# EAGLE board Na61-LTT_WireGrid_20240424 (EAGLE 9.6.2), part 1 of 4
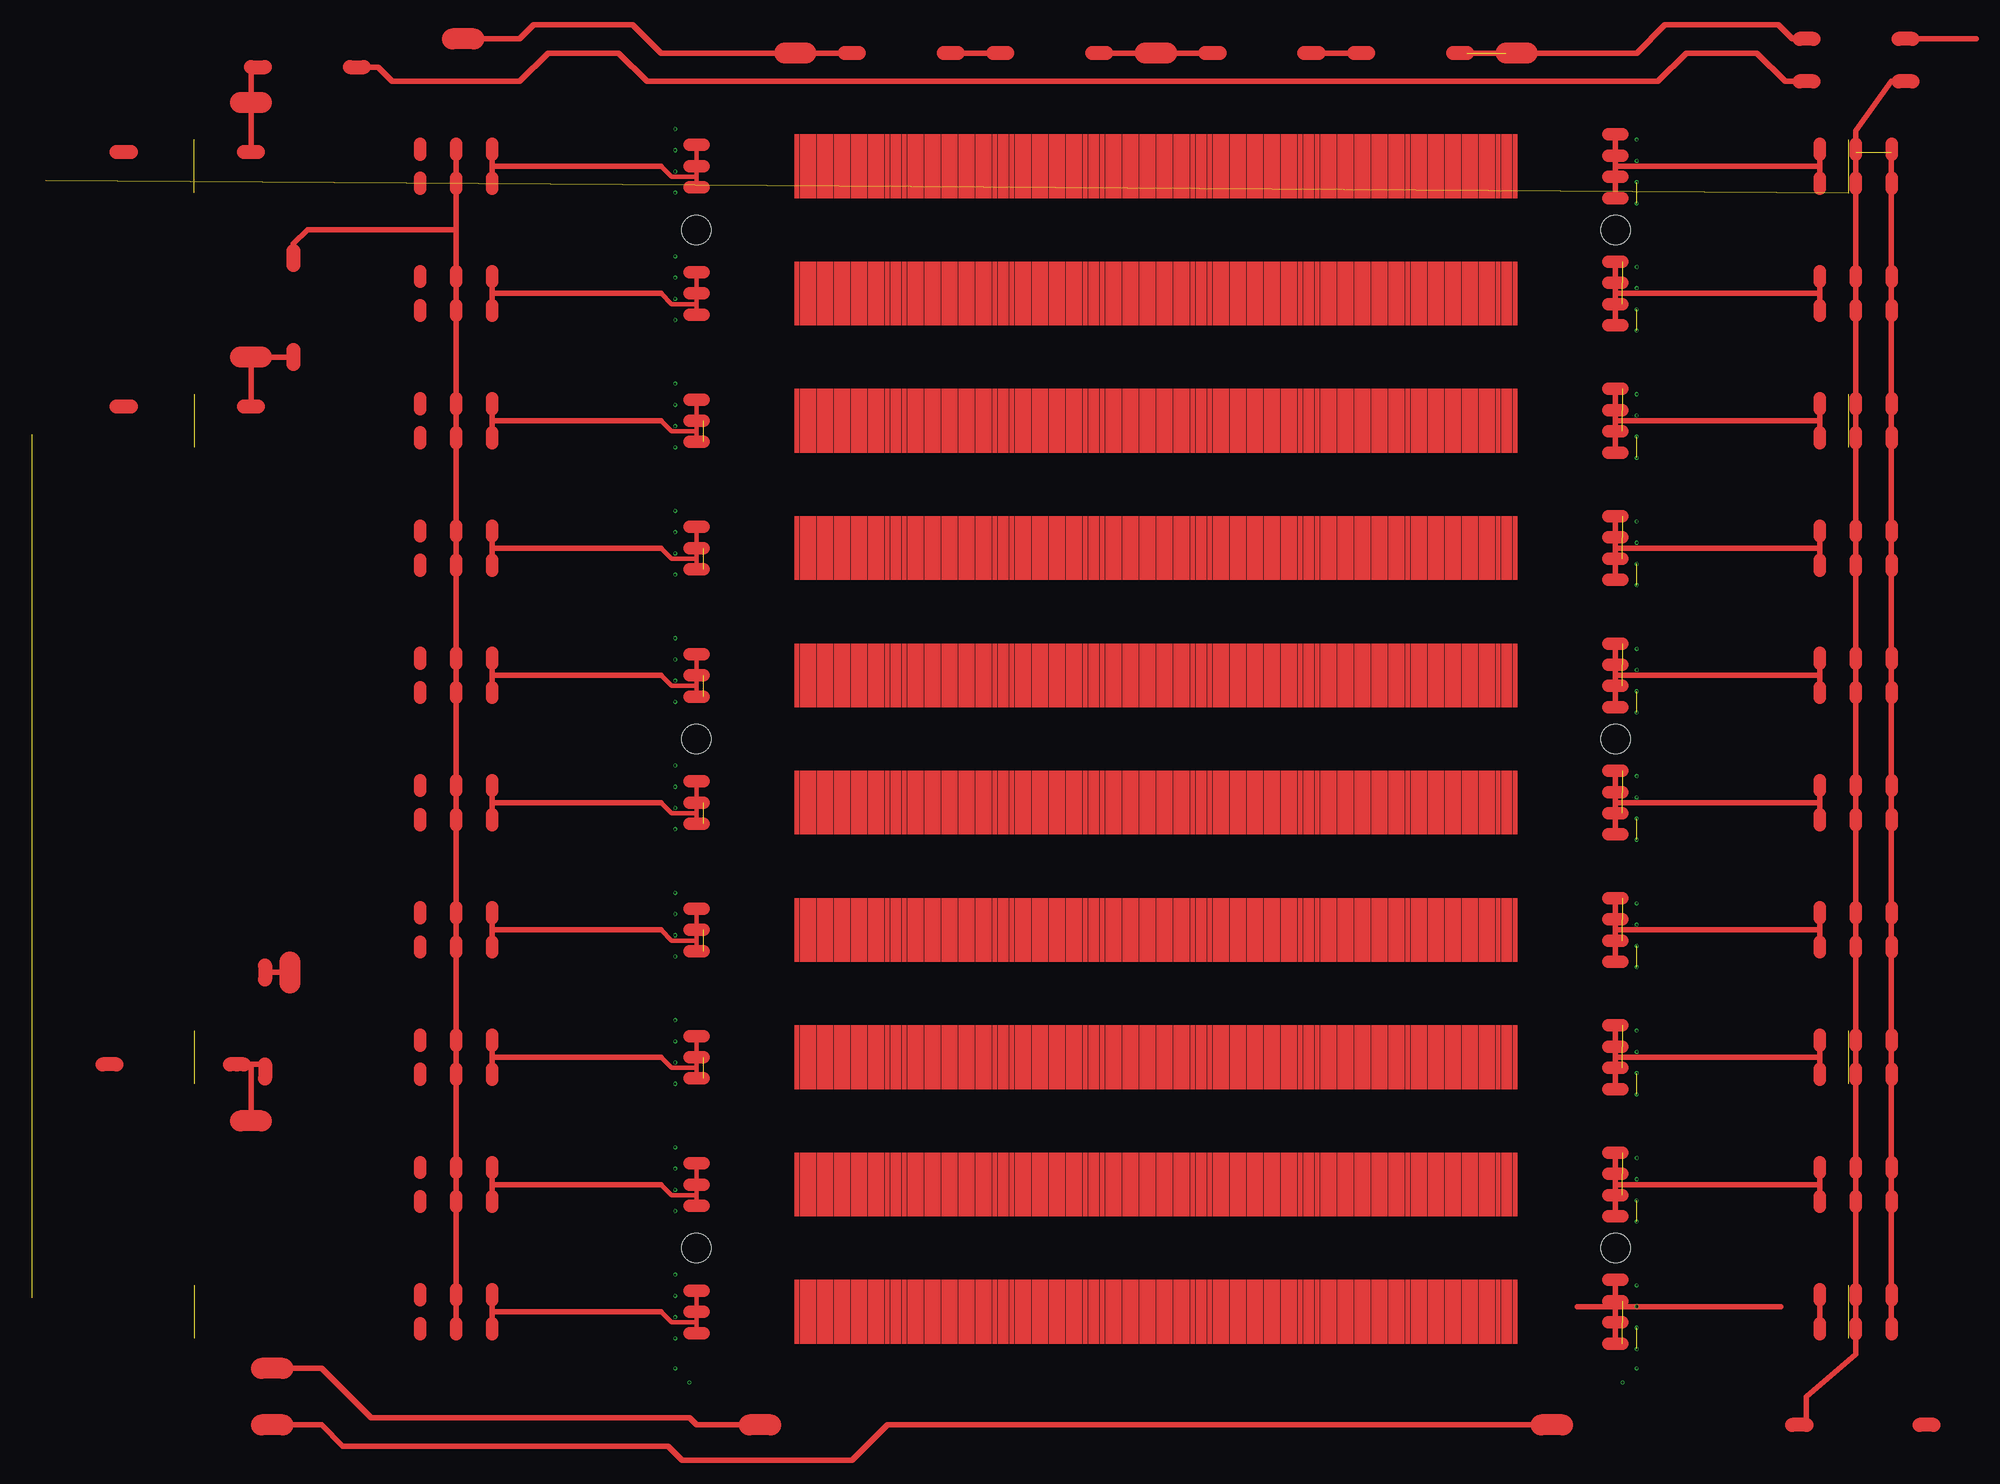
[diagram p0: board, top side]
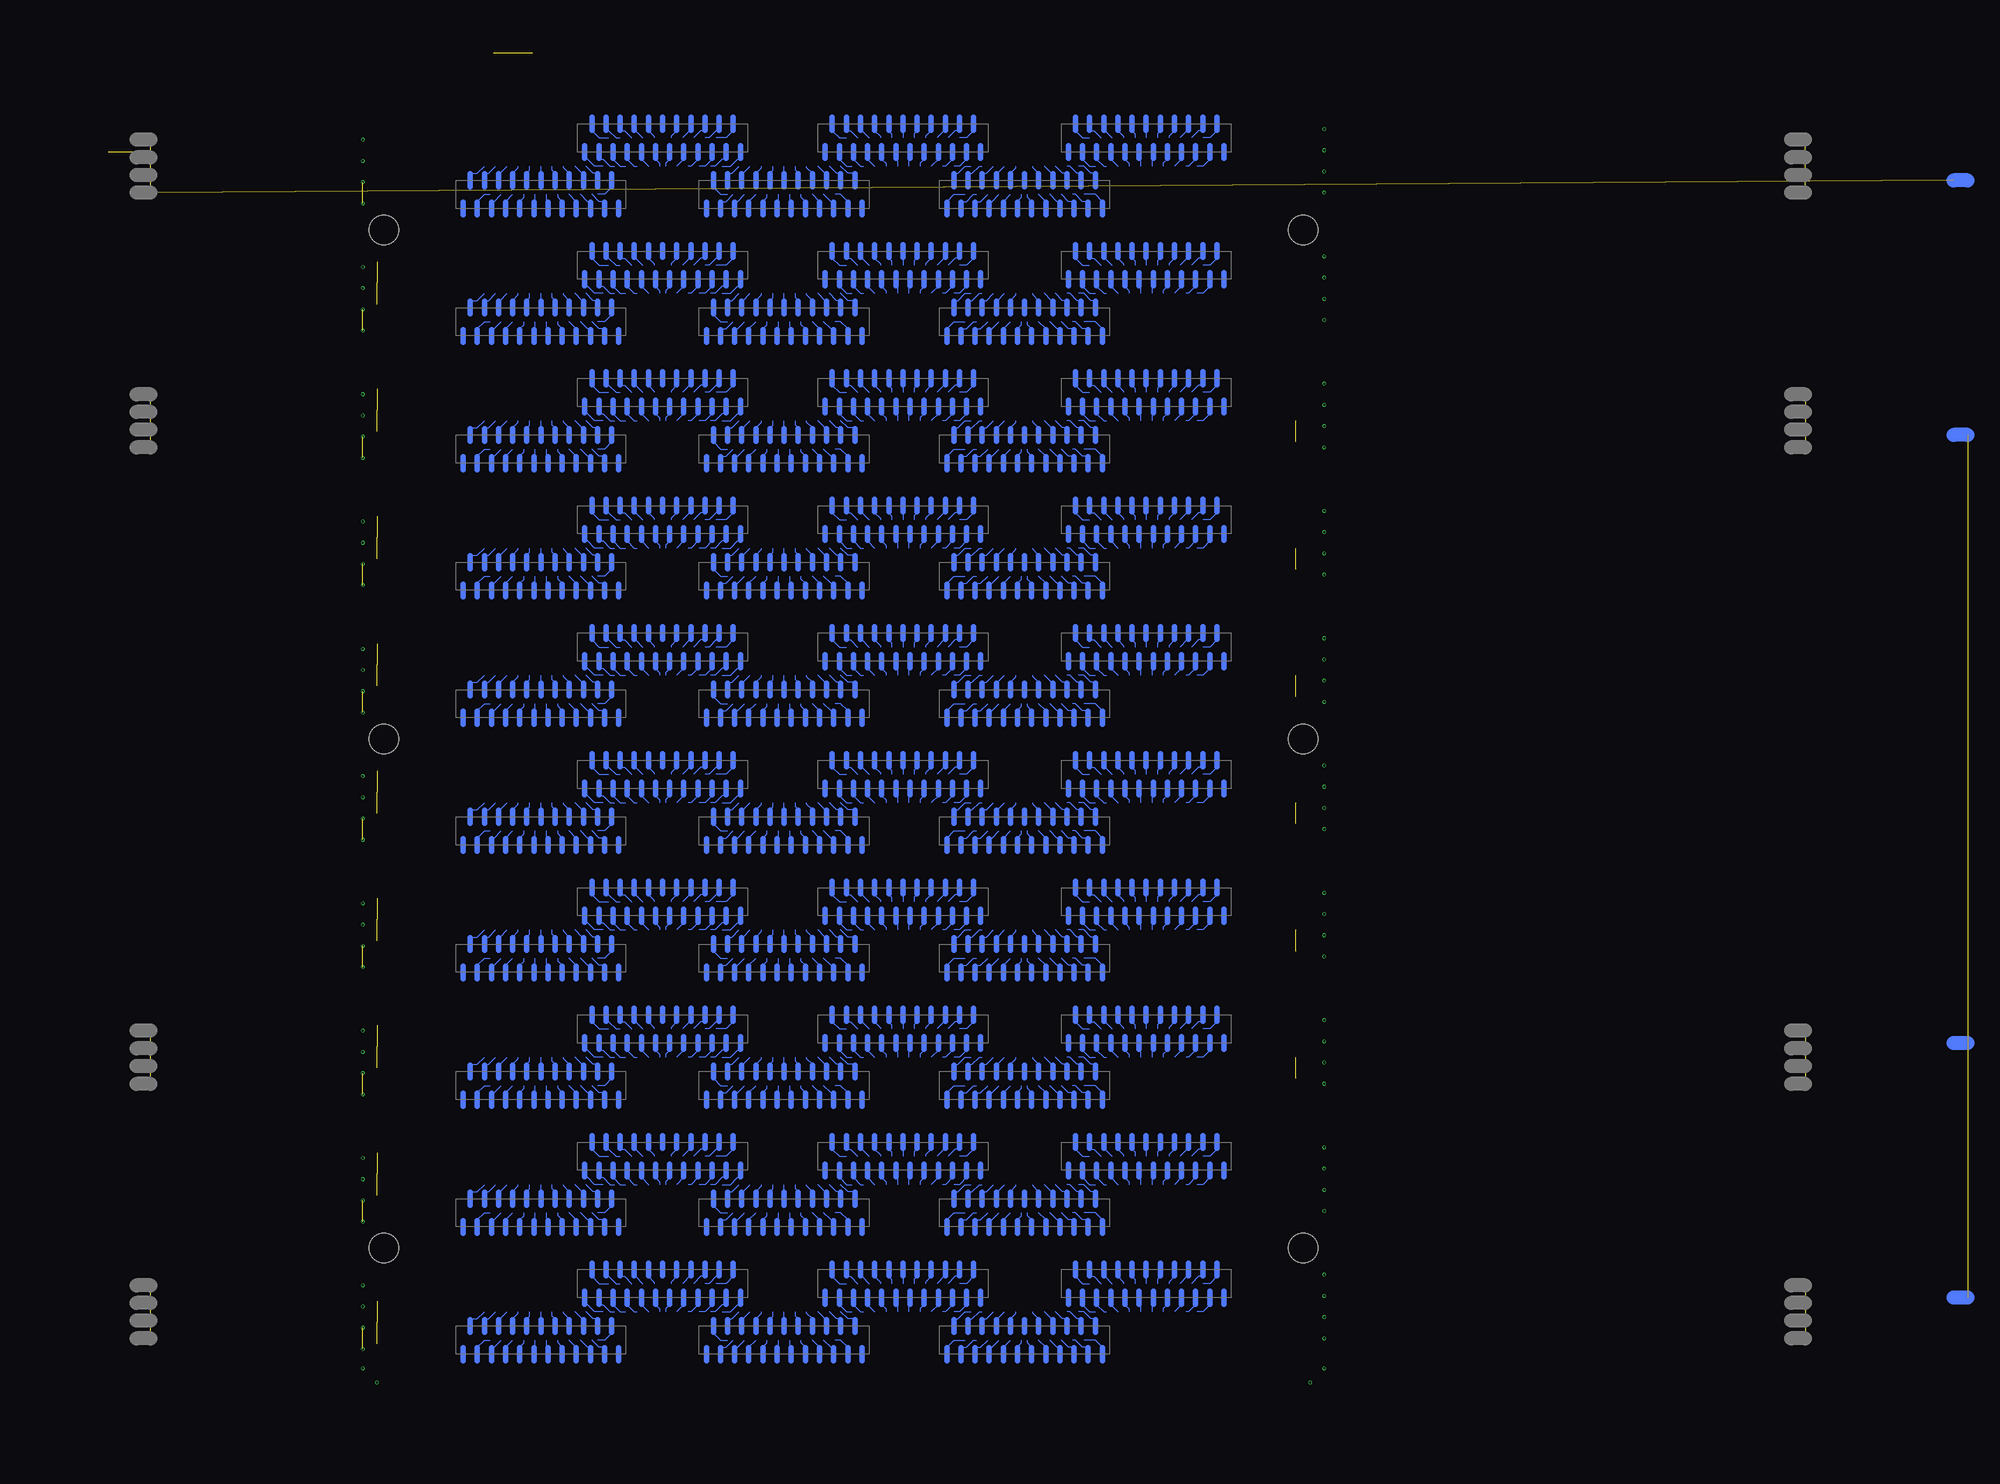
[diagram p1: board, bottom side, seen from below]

No outline drawn. Coordinates in mm, seen from the top.
Copper layers (1*16): Top 0.035mm / dielectric 1.5mm / Bottom 0.035mm
Design rules "default *": minimum track width 6mil, minimum drill 0.2mm, track to track 6mil, track to pad 6mil, pad to pad 6mil, via to via 6mil, smd to smd 6mil, copper to edge 40mil, drill to drill 6mil, minimum pad ring 8mil, minimum via ring 4mil, stop-mask expansion 4mil, vias tented up to drill 0mil, thermal gap 10mil
Holes 4.2 mm at -65,153 65,153 -65,9 65,9 -65,81 65,81

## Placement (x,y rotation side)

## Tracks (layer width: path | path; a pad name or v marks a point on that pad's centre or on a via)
S$1
  Bottom 0.8: 11.4,-5.1 11.4,-6.9
S$2
  Bottom 0.8: 10.4,-2.9 10.4,-1.1
S$3
  Bottom 0.8: 7.4,-5.1 7.4,-6.9
S$4
  Bottom 0.8: 4.4,-2.9 4.4,-1.1
S$5
  Bottom 0.8: 1.4,-5.1 1.4,-6.9
S$6
  Bottom 0.8: 0.4,-2.9 0.4,-1.1
S$7
  Bottom 0.8: -2.6,-5.1 -2.6,-6.9
S$8
  Bottom 0.8: -1.6,-2.9 -1.6,-1.1
S$9
  Bottom 0.8: 19.4,-5.1 19.4,-6.9
S$10
  Bottom 0.8: 18.4,-2.9 18.4,-1.1
S$11
  Bottom 0.8: 15.4,-5.1 15.4,-6.9
S$12
  Bottom 0.8: 14.4,-2.9 14.4,-1.1
S$13
  Bottom 0.8: 16.4,-2.9 16.4,-1.1
S$14
  Bottom 0.8: 17.4,-5.1 17.4,-6.9
S$15
  Bottom 0.8: 13.4,-5.1 13.4,-6.9
S$16
  Bottom 0.8: 12.4,-2.9 12.4,-1.1
S$17
  Bottom 0.8: 8.4,-2.9 8.4,-1.1
S$18
  Bottom 0.8: 9.4,-5.1 9.4,-6.9
S$19
  Bottom 0.8: 5.4,-5.1 5.4,-6.9
S$20
  Bottom 0.8: 6.4,-2.9 6.4,-1.1
S$21
  Bottom 0.8: 2.4,-2.9 2.4,-1.1
S$22
  Bottom 0.8: 3.4,-5.1 3.4,-6.9
S$23
  Bottom 0.8: -0.6,-5.1 -0.6,-6.9
S$24
  Bottom 0.8: -7.4,2.9 -7.4,1.1
S$25
  Bottom 0.8: -5.4,2.9 -5.4,1.1
S$26
  Bottom 0.8: -8.4,5.1 -8.4,6.9
S$27
  Bottom 0.8: -6.4,5.1 -6.4,6.9
S$28
  Bottom 0.8: -11.4,2.9 -11.4,1.1
S$29
  Bottom 0.8: -9.4,2.9 -9.4,1.1
S$30
  Bottom 0.8: -10.4,5.1 -10.4,6.9
S$31
  Bottom 0.8: -12.4,5.1 -12.4,6.9
S$32
  Bottom 0.8: -13.4,2.9 -13.4,1.1
S$33
  Bottom 0.8: -15.4,2.9 -15.4,1.1
S$34
  Bottom 0.8: -14.4,5.1 -14.4,6.9
S$35
  Bottom 0.8: -16.4,5.1 -16.4,6.9
S$36
  Bottom 0.8: -17.4,2.9 -17.4,1.1
S$37
  Bottom 0.8: -19.4,2.9 -19.4,1.1
S$38
  Bottom 0.8: -18.4,5.1 -18.4,6.9
S$39
  Bottom 0.8: 0.6,2.9 0.6,1.1
S$40
  Bottom 0.8: 2.6,2.9 2.6,1.1
S$41
  Bottom 0.8: -0.4,5.1 -0.4,6.9
S$42
  Bottom 0.8: 1.6,5.1 1.6,6.9
S$43
  Bottom 0.8: -3.4,2.9 -3.4,1.1
S$44
  Bottom 0.8: -1.4,2.9 -1.4,1.1
S$45
  Bottom 0.8: -4.4,5.1 -4.4,6.9
S$46
  Bottom 0.8: -2.4,5.1 -2.4,6.9
S$47
  Bottom 0.8: -24.6,-5.1 -24.6,-6.9
S$48
  Bottom 0.8: -22.6,-5.1 -22.6,-6.9
S$49
  Bottom 0.8: -25.6,-2.9 -25.6,-1.1
S$50
  Bottom 0.8: -23.6,-2.9 -23.6,-1.1
S$51
  Bottom 0.8: -28.6,-5.1 -28.6,-6.9
S$52
  Bottom 0.8: -26.6,-5.1 -26.6,-6.9
S$53
  Bottom 0.8: -27.6,-2.9 -27.6,-1.1
S$54
  Bottom 0.8: -29.6,-2.9 -29.6,-1.1
S$55
  Bottom 0.8: -30.6,-5.1 -30.6,-6.9
S$56
  Bottom 0.8: -32.6,-5.1 -32.6,-6.9
S$57
  Bottom 0.8: -31.6,-2.9 -31.6,-1.1
S$58
  Bottom 0.8: -33.6,-2.9 -33.6,-1.1
S$59
  Bottom 0.8: -34.6,-5.1 -34.6,-6.9
S$60
  Bottom 0.8: -36.6,-5.1 -36.6,-6.9
S$61
  Bottom 0.8: -35.6,-2.9 -35.6,-1.1
S$62
  Bottom 0.8: -16.6,-5.1 -16.6,-6.9
S$63
  Bottom 0.8: -14.6,-5.1 -14.6,-6.9
S$64
  Bottom 0.8: -17.6,-2.9 -17.6,-1.1
S$65
  Bottom 0.8: -15.6,-2.9 -15.6,-1.1
S$66
  Bottom 0.8: -20.6,-5.1 -20.6,-6.9
S$67
  Bottom 0.8: -18.6,-5.1 -18.6,-6.9
S$68
  Bottom 0.8: -21.6,-2.9 -21.6,-1.1
S$69
  Bottom 0.8: -19.6,-2.9 -19.6,-1.1
S$70
  Bottom 0.8: 26.6,2.9 26.6,1.1
S$71
  Bottom 0.8: 28.6,2.9 28.6,1.1
S$72
  Bottom 0.8: 25.6,5.1 25.6,6.9
S$73
  Bottom 0.8: 27.6,5.1 27.6,6.9
S$74
  Bottom 0.8: 22.6,2.9 22.6,1.1
S$75
  Bottom 0.8: 24.6,2.9 24.6,1.1
S$76
  Bottom 0.8: 23.6,5.1 23.6,6.9
S$77
  Bottom 0.8: 21.6,5.1 21.6,6.9
S$78
  Bottom 0.8: 20.6,2.9 20.6,1.1
S$79
  Bottom 0.8: 18.6,2.9 18.6,1.1
S$80
  Bottom 0.8: 19.6,5.1 19.6,6.9
S$81
  Bottom 0.8: 17.6,5.1 17.6,6.9
S$82
  Bottom 0.8: 16.6,2.9 16.6,1.1
S$83
  Bottom 0.8: 14.6,2.9 14.6,1.1
S$84
  Bottom 0.8: 15.6,5.1 15.6,6.9
S$85
  Bottom 0.8: 34.6,2.9 34.6,1.1
S$86
  Bottom 0.8: 36.6,2.9 36.6,1.1
S$87
  Bottom 0.8: 33.6,5.1 33.6,6.9
S$88
  Bottom 0.8: 35.6,5.1 35.6,6.9
S$89
  Bottom 0.8: 30.6,2.9 30.6,1.1
S$90
  Bottom 0.8: 32.6,2.9 32.6,1.1
S$91
  Bottom 0.8: 29.6,5.1 29.6,6.9
S$92
  Bottom 0.8: 31.6,5.1 31.6,6.9
S$93
  Bottom 0.8: -41.8,2.9 -41.8,1.1
S$94
  Bottom 0.8: -39.8,2.9 -39.8,1.1
S$95
  Bottom 0.8: -42.8,5.1 -42.8,6.9
S$96
  Bottom 0.8: -40.8,5.1 -40.8,6.9
S$97
  Bottom 0.8: -45.8,2.9 -45.8,1.1
S$98
  Bottom 0.8: -43.8,2.9 -43.8,1.1
S$99
  Bottom 0.8: -44.8,5.1 -44.8,6.9
S$100
  Bottom 0.8: -46.8,5.1 -46.8,6.9
S$101
  Bottom 0.8: -47.8,2.9 -47.8,1.1
S$102
  Bottom 0.8: -49.8,2.9 -49.8,1.1
S$103
  Bottom 0.8: -48.8,5.1 -48.8,6.9
S$104
  Bottom 0.8: -50.8,5.1 -50.8,6.9
S$105
  Bottom 0.8: -51.8,2.9 -51.8,1.1
S$106
  Bottom 0.8: -53.8,2.9 -53.8,1.1
S$107
  Bottom 0.8: -52.8,5.1 -52.8,6.9
S$108
  Bottom 0.8: -33.8,2.9 -33.8,1.1
S$109
  Bottom 0.8: -31.8,2.9 -31.8,1.1
S$110
  Bottom 0.8: -34.8,5.1 -34.8,6.9
S$111
  Bottom 0.8: -32.8,5.1 -32.8,6.9
S$112
  Bottom 0.8: -37.8,2.9 -37.8,1.1
S$113
  Bottom 0.8: -35.8,2.9 -35.8,1.1
S$114
  Bottom 0.8: -38.8,5.1 -38.8,6.9
S$115
  Bottom 0.8: -36.8,5.1 -36.8,6.9
S$116
  Bottom 0.8: 43.8,-5.1 43.8,-6.9
S$117
  Bottom 0.8: 45.8,-5.1 45.8,-6.9
S$118
  Bottom 0.8: 42.8,-2.9 42.8,-1.1
S$119
  Bottom 0.8: 44.8,-2.9 44.8,-1.1
S$120
  Bottom 0.8: 39.8,-5.1 39.8,-6.9
S$121
  Bottom 0.8: 41.8,-5.1 41.8,-6.9
S$122
  Bottom 0.8: 40.8,-2.9 40.8,-1.1
S$123
  Bottom 0.8: 38.8,-2.9 38.8,-1.1
S$124
  Bottom 0.8: 37.8,-5.1 37.8,-6.9
S$125
  Bottom 0.8: 35.8,-5.1 35.8,-6.9
S$126
  Bottom 0.8: 36.8,-2.9 36.8,-1.1
S$127
  Bottom 0.8: 34.8,-2.9 34.8,-1.1
S$128
  Bottom 0.8: 33.8,-5.1 33.8,-6.9
S$129
  Bottom 0.8: 31.8,-5.1 31.8,-6.9
S$130
  Bottom 0.8: 32.8,-2.9 32.8,-1.1
S$131
  Bottom 0.8: 51.8,-5.1 51.8,-6.9
S$132
  Bottom 0.8: 53.8,-5.1 53.8,-6.9
S$133
  Bottom 0.8: 50.8,-2.9 50.8,-1.1
S$134
  Bottom 0.8: 52.8,-2.9 52.8,-1.1
S$135
  Bottom 0.8: 47.8,-5.1 47.8,-6.9
S$136
  Bottom 0.8: 49.8,-5.1 49.8,-6.9
S$137
  Bottom 0.8: 46.8,-2.9 46.8,-1.1
S$138
  Bottom 0.8: 48.8,-2.9 48.8,-1.1
S$139
  Top 0.61: -65,3 -65,-1.5 | -65,-1.5 -65,-3 | -65,-1.5 -68.5,-1.5 -70,0
  Top 0.813: -70,0 -93.5,0
  Top 1.8: -64,3 -65,3 -66,3 | -64,-3 -65,-3 -66,-3
S$140
  Top 1.778: -104.08,1.65 -104.08,3.17
S$141  (via drill 0.3)  (1 unrouted)
  other vias: 68,-2.25 68,-5.25
S$142
  Top 1.778: -99,1.65 -99,3.17
S$143
  Top 1.778: -93.92,1.65 -93.92,3.17
S$144
  Top 1.778: 93.92,-3.17 93.92,-1.65
S$145
  Bottom 0.8: 9.4,12.9 9.4,11.1
S$146
  Top 1.778: 93.92,1.65 93.92,3.17
S$147
  Top 1.778: 99,-3.17 99,-1.65
S$148
  Top 1.778: 99,1.65 99,3.17
S$149
  Top 1.778: 104.08,-3.17 104.08,-1.65
S$150
  Top 1.778: 104.08,1.65 104.08,3.17
S$151  (via drill 0.3)
  other vias: 68,3.75
S$152  (via drill 0.3)
  other vias: -68,-3.75
S$153  (via drill 0.3)
  other vias: -68,-0.75
S$154  (via drill 0.3)
  other vias: -68,2.25
S$155  (via drill 0.3)
  other vias: -68,5.25
S$156  (via drill 0.3)
  other vias: 68,18.75
S$157  (via drill 0.3)  (1 unrouted)
  other vias: 68,15.75 68,12.75
S$158
  Bottom 0.8: 11.4,12.9 11.4,11.1
S$159
  Bottom 0.8: 8.4,15.1 8.4,16.9
S$160
  Bottom 0.8: 10.4,15.1 10.4,16.9
S$161
  Bottom 0.8: 5.4,12.9 5.4,11.1
S$162  (via drill 0.3)
  other vias: 68,21.75
S$163  (via drill 0.3)
  other vias: -68,14.25
S$164  (via drill 0.3)
  other vias: -68,17.25
S$165  (via drill 0.3)
  other vias: -68,20.25
S$166  (via drill 0.3)
  other vias: -68,23.25
S$167  (via drill 0.3)
  other vias: 68,36.75
S$168  (via drill 0.3)  (1 unrouted)
  other vias: 68,33.75 68,30.75
S$169  (via drill 0.3)
  other vias: 68,39.75
S$170  (via drill 0.3)
  other vias: -68,32.25
S$171  (via drill 0.3)
  other vias: -68,35.25
S$172  (via drill 0.3)
  other vias: -68,38.25
S$173  (via drill 0.3)
  other vias: -68,41.25
S$174  (via drill 0.3)
  other vias: 68,54.75
S$175  (via drill 0.3)  (1 unrouted)
  other vias: 68,51.75 68,48.75
S$176  (via drill 0.3)
  other vias: 68,57.75
S$177  (via drill 0.3)
  other vias: -68,50.25
S$178  (via drill 0.3)
  other vias: -68,53.25
S$179  (via drill 0.3)
  other vias: -68,56.25
S$180  (via drill 0.3)
  other vias: -68,59.25
S$181  (via drill 0.3)
  other vias: 68,72.75
S$182  (via drill 0.3)  (1 unrouted)
  other vias: 68,69.75 68,66.75
S$183  (via drill 0.3)
  other vias: 68,75.75
S$184  (via drill 0.3)
  other vias: -68,68.25
S$185  (via drill 0.3)
  other vias: -68,71.25
S$186  (via drill 0.3)
  other vias: -68,74.25
S$187  (via drill 0.3)
  other vias: -68,77.25
S$188  (via drill 0.3)
  other vias: 68,90.75
S$189  (via drill 0.3)  (1 unrouted)
  other vias: 68,87.75 68,84.75
S$190  (via drill 0.3)
  other vias: 68,93.75
S$191  (via drill 0.3)
  other vias: -68,86.25
S$192  (via drill 0.3)
  other vias: -68,89.25
S$193  (via drill 0.3)
  other vias: -68,92.25
S$194  (via drill 0.3)
  other vias: -68,95.25
S$195  (via drill 0.3)
  other vias: 68,108.75
S$196  (via drill 0.3)  (1 unrouted)
  other vias: 68,105.75 68,102.75
S$197  (via drill 0.3)
  other vias: 68,111.75
S$198  (via drill 0.3)
  other vias: -68,104.25
S$199  (via drill 0.3)
  other vias: -68,107.25
S$200  (via drill 0.3)
  other vias: -68,110.25
S$201  (via drill 0.3)
  other vias: -68,113.25
S$202  (via drill 0.3)
  other vias: 68,126.75
S$203  (via drill 0.3)  (1 unrouted)
  other vias: 68,123.75 68,120.75
S$204  (via drill 0.3)
  other vias: 68,129.75
S$205  (via drill 0.3)
  other vias: -68,122.25
S$206  (via drill 0.3)
  other vias: -68,125.25
S$207  (via drill 0.3)
  other vias: -68,128.25
S$208  (via drill 0.3)
  other vias: -68,131.25
S$209  (via drill 0.3)
  other vias: 68,144.75
S$210  (via drill 0.3)  (1 unrouted)
  other vias: 68,141.75 68,138.75
S$211  (via drill 0.3)
  other vias: 68,147.75
S$212  (via drill 0.3)
  other vias: -68,140.25
S$213  (via drill 0.3)
  other vias: -68,143.25
S$214  (via drill 0.3)
  other vias: -68,146.25
S$215  (via drill 0.3)
  other vias: -68,149.25
S$216  (via drill 0.3)
  other vias: 68,162.75
S$217  (via drill 0.3)  (1 unrouted)
  other vias: 68,159.75 68,156.75
S$218  (via drill 0.3)
  other vias: 68,165.75
S$219  (via drill 0.3)
  other vias: -68,158.25
S$220  (via drill 0.3)
  other vias: -68,161.25
S$221  (via drill 0.3)
  other vias: -68,164.25
S$222  (via drill 0.3)
  other vias: -68,167.25
S$223  (via drill 0.3)
  other vias: -68,-8
S$224  (via drill 0.3)
  other vias: 68,-8
S$225  (via drill 0.3)
  other vias: 66,-10
S$226  (via drill 0.3)
  other vias: -66,-10
S$290
  Bottom 0.152: -52.8,5 -51.8,4
S$291
  Bottom 0.152: -51.8,4 -50.8,4
S$292
  Bottom 0.152: -50.8,5 -50.2,5
S$293
  Bottom 0.152: -50.2,5 -49.2,4
S$294
  Bottom 0.152: -48.8,5 -48.6,5
S$295
  Bottom 0.152: -48.6,5 -47.6,4
S$296
  Bottom 0.152: -46.8,5 -46,4.2
S$297
  Bottom 0.152: -46,4.2 -46,4
S$298
  Bottom 0.152: -44.8,5 -44.4,4.6
S$299
  Bottom 0.152: -44.4,4.6 -44.4,4
S$300
  Bottom 0.152: -42.8,5 -42.8,4
S$301
  Bottom 0.152: -40.8,5 -41.2,4.6
S$302
  Bottom 0.152: -41.2,4.6 -41.2,4
S$303
  Bottom 0.152: -38.8,5 -39.6,4.2
S$304
  Bottom 0.152: -39.6,4.2 -39.6,4
S$305
  Bottom 0.152: -36.8,5 -37,5
S$306
  Bottom 0.152: -37,5 -38,4
S$307
  Bottom 0.152: -34.8,5 -35.4,5
S$308
  Bottom 0.152: -35.4,5 -36.4,4
S$309
  Bottom 0.152: -32.8,5 -33.8,4
S$310
  Bottom 0.152: -33.8,4 -34.8,4
S$311
  Bottom 0.152: -51.8,1 -50.8,0
S$312
  Bottom 0.152: -50.8,0 -50,0
S$313
  Bottom 0.152: -49.8,1 -48.8,0
S$314
  Bottom 0.152: -48.8,0 -48.4,0
S$315
  Bottom 0.152: -47.8,1 -46.8,0
S$316
  Bottom 0.152: -45.8,1 -45.2,0.4
S$317
  Bottom 0.152: -45.2,0.4 -45.2,0
S$318
  Bottom 0.152: -43.8,1 -43.6,0.8
S$319
  Bottom 0.152: -43.6,0.8 -43.6,0
S$320
  Bottom 0.152: -41.8,1 -42,0.8
S$321
  Bottom 0.152: -42,0.8 -42,0
S$322
  Bottom 0.152: -39.8,1 -40.4,0.4
S$323
  Bottom 0.152: -40.4,0.4 -40.4,0
S$324
  Bottom 0.152: -37.8,1 -38.8,0
S$325
  Bottom 0.152: -35.8,1 -36.8,0
S$326
  Bottom 0.152: -36.8,0 -37.2,0
S$327
  Bottom 0.152: -33.8,1 -34.8,0
S$328
  Bottom 0.152: -34.8,0 -35.6,0
S$329
  Bottom 0.152: -36.6,-5 -35.6,-4
S$330
  Bottom 0.152: -35.6,-4 -34,-4
S$331
  Bottom 0.152: -34.6,-5 -33.8,-5
S$332
  Bottom 0.152: -33.8,-5 -32.8,-4
S$333
  Bottom 0.152: -32.8,-4 -32.4,-4
S$334
  Bottom 0.152: -32.6,-5 -31.8,-5
S$335
  Bottom 0.152: -31.8,-5 -30.8,-4
S$336
  Bottom 0.152: -30.6,-5 -30.2,-5
S$337
  Bottom 0.152: -30.2,-5 -29.2,-4
S$338
  Bottom 0.152: -28.6,-5 -27.6,-4
S$339
  Bottom 0.152: -26.6,-5 -26,-4.4
S$340
  Bottom 0.152: -26,-4.4 -26,-4
S$341
  Bottom 0.152: -35.6,-1 -35,-1
S$342
  Bottom 0.152: -35,-1 -34,0
S$343
  Bottom 0.152: -34,0 -33.2,0
S$344
  Bottom 0.152: -33.6,-1 -33,-1
S$345
  Bottom 0.152: -33,-1 -32,0
S$346
  Bottom 0.152: -32,0 -31.6,0
S$347
  Bottom 0.152: -31.6,-1 -31,-1
S$348
  Bottom 0.152: -31,-1 -30,0
S$349
  Bottom 0.152: -29.6,-1 -29.4,-1
S$350
  Bottom 0.152: -29.4,-1 -28.4,0
S$351
  Bottom 0.152: -27.6,-1 -26.8,-0.2
S$352
  Bottom 0.152: -26.8,-0.2 -26.8,0
S$353
  Bottom 0.152: 1.6,5 0.6,4
S$354
  Bottom 0.152: 0.6,4 -0.4,4
S$355
  Bottom 0.152: -0.4,5 -1,5
S$356
  Bottom 0.152: -1,5 -2,4
S$357
  Bottom 0.152: -2.4,5 -2.6,5
S$358
  Bottom 0.152: -2.6,5 -3.6,4
S$359
  Bottom 0.152: -4.4,5 -5.2,4.2
S$360
  Bottom 0.152: -5.2,4.2 -5.2,4
S$361
  Bottom 0.152: -6.4,5 -6.8,4.6
S$362
  Bottom 0.152: -6.8,4.6 -6.8,4
S$363
  Bottom 0.152: -8.4,5 -8.4,4
S$364
  Bottom 0.152: -10.4,5 -10,4.6
S$365
  Bottom 0.152: -10,4.6 -10,4
S$366
  Bottom 0.152: -12.4,5 -11.6,4.2
S$367
  Bottom 0.152: -11.6,4.2 -11.6,4
S$368
  Bottom 0.152: -14.4,5 -14.2,5
S$369
  Bottom 0.152: -14.2,5 -13.2,4
S$370
  Bottom 0.152: -16.4,5 -15.8,5
S$371
  Bottom 0.152: -15.8,5 -14.8,4
S$372
  Bottom 0.152: -18.4,5 -17.4,4
S$373
  Bottom 0.152: -17.4,4 -16.4,4
S$374
  Bottom 0.152: 0.6,1 -0.4,0
S$375
  Bottom 0.152: -0.4,0 -1.2,0
S$376
  Bottom 0.152: -1.4,1 -2.4,0
S$377
  Bottom 0.152: -2.4,0 -2.8,0
S$378
  Bottom 0.152: -3.4,1 -4.4,0
S$379
  Bottom 0.152: -5.4,1 -6,0.4
S$380
  Bottom 0.152: -6,0.4 -6,0
S$381
  Bottom 0.152: -7.4,1 -7.6,0.8
S$382
  Bottom 0.152: -7.6,0.8 -7.6,0
S$383
  Bottom 0.152: -9.4,1 -9.2,0.8
S$384
  Bottom 0.152: -9.2,0.8 -9.2,0
S$385
  Bottom 0.152: -11.4,1 -10.8,0.4
S$386
  Bottom 0.152: -10.8,0.4 -10.8,0
S$387
  Bottom 0.152: -13.4,1 -12.4,0
S$388
  Bottom 0.152: -15.4,1 -14.4,0
S$389
  Bottom 0.152: -14.4,0 -14,0
S$390
  Bottom 0.152: -17.4,1 -16.4,0
S$391
  Bottom 0.152: -16.4,0 -15.6,0
S$392
  Bottom 0.152: -14.6,-5 -15.6,-4
S$393
  Bottom 0.152: -15.6,-4 -17.2,-4
S$394
  Bottom 0.152: -16.6,-5 -17.4,-5
S$395
  Bottom 0.152: -17.4,-5 -18.4,-4
S$396
  Bottom 0.152: -18.4,-4 -18.8,-4
S$397
  Bottom 0.152: -18.6,-5 -19.4,-5
S$398
  Bottom 0.152: -19.4,-5 -20.4,-4
S$399
  Bottom 0.152: -20.6,-5 -21,-5
S$400
  Bottom 0.152: -21,-5 -22,-4
S$401
  Bottom 0.152: -22.6,-5 -23.6,-4
S$402
  Bottom 0.152: -24.6,-5 -25.2,-4.4
S$403
  Bottom 0.152: -25.2,-4.4 -25.2,-4
S$404
  Bottom 0.152: -15.6,-1 -16.2,-1
S$405
  Bottom 0.152: -16.2,-1 -17.2,0
S$406
  Bottom 0.152: -17.2,0 -18,0
S$407
  Bottom 0.152: -17.6,-1 -18.2,-1
S$408
  Bottom 0.152: -18.2,-1 -19.2,0
S$409
  Bottom 0.152: -19.2,0 -19.6,0
S$410
  Bottom 0.152: -19.6,-1 -20.2,-1
S$411
  Bottom 0.152: -20.2,-1 -21.2,0
S$412
  Bottom 0.152: -21.6,-1 -21.8,-1
S$413
  Bottom 0.152: -21.8,-1 -22.8,0
S$414
  Bottom 0.152: -23.6,-1 -24.4,-0.2
S$415
  Bottom 0.152: -24.4,-0.2 -24.4,0
S$416
  Bottom 0.152: 0.4,-1 1,-1
S$417
  Bottom 0.152: 1,-1 2,0
S$418
  Bottom 0.152: 2.4,-1 2.6,-1
S$419
  Bottom 0.152: 2.6,-1 3.6,0
S$420
  Bottom 0.152: 4.4,-1 5.2,-0.2
S$421
  Bottom 0.152: 5.2,-0.2 5.2,0
S$422
  Bottom 0.152: 6.4,-1 6.8,-0.6
S$423
  Bottom 0.152: 6.8,-0.6 6.8,0
S$424
  Bottom 0.152: 8.4,-1 8.4,0
S$425
  Bottom 0.152: -1.6,-1 -0.6,-1
S$426
  Bottom 0.152: -0.6,-1 0.4,0
S$427
  Bottom 0.152: -0.6,-5 0.4,-4
S$428
  Bottom 0.152: 0.4,-4 1.2,-4
S$429
  Bottom 0.152: 1.4,-5 1.8,-5
S$430
  Bottom 0.152: 1.8,-5 2.8,-4
S$431
  Bottom 0.152: 3.4,-5 4.4,-4
S$432
  Bottom 0.152: 5.4,-5 6,-4.4
S$433
  Bottom 0.152: 6,-4.4 6,-4
S$434
  Bottom 0.152: 7.4,-5 7.6,-4.8
S$435
  Bottom 0.152: 7.6,-4.8 7.6,-4
S$436
  Bottom 0.152: 9.4,-5 9.2,-4.8
S$437
  Bottom 0.152: 9.2,-4.8 9.2,-4
S$438
  Bottom 0.152: 11.4,-5 10.8,-4.4
S$439
  Bottom 0.152: 10.8,-4.4 10.8,-4
S$440
  Bottom 0.152: 13.4,-5 12.4,-4
S$441
  Bottom 0.152: 15.4,-5 15,-5
S$442
  Bottom 0.152: 15,-5 14,-4
S$443
  Bottom 0.152: 17.4,-5 16.6,-5
S$444
  Bottom 0.152: 16.6,-5 15.6,-4
S$445
  Bottom 0.152: 10.4,-1 10,-0.6
S$446
  Bottom 0.152: 10,-0.6 10,0
S$447
  Bottom 0.152: 12.4,-1 11.6,-0.2
S$448
  Bottom 0.152: 11.6,-0.2 11.6,0
S$449
  Bottom 0.152: 14.4,-1 14.2,-1
S$450
  Bottom 0.152: 14.2,-1 13.2,0
S$451
  Bottom 0.152: 16.4,-1 15.8,-1
S$452
  Bottom 0.152: 15.8,-1 14.8,0
S$453
  Bottom 0.152: 18.4,-3 17.4,-4
S$454
  Bottom 0.152: 17.4,-4 16.4,-4
S$455
  Bottom 0.152: 16.6,1 17.2,1
S$456
  Bottom 0.152: 17.2,1 18.2,0
S$457
  Bottom 0.152: 18.2,0 18.8,0
S$458
  Bottom 0.152: 18.6,1 19.6,0
S$459
  Bottom 0.152: 19.6,0 20.4,0
S$460
  Bottom 0.152: 20.6,1 21.6,0
S$461
  Bottom 0.152: 21.6,0 22,0
S$462
  Bottom 0.152: 22.6,1 23.6,0
S$463
  Bottom 0.152: 24.6,1 25.2,0.4
S$464
  Bottom 0.152: 25.2,0.4 25.2,0
S$465
  Bottom 0.152: 15.6,5 16.6,4
S$466
  Bottom 0.152: 16.6,4 18,4
S$467
  Bottom 0.152: 17.6,5 18,5
S$468
  Bottom 0.152: 18,5 19,4
S$469
  Bottom 0.152: 19,4 19.6,4
S$470
  Bottom 0.152: 19.6,5 20.2,5
S$471
  Bottom 0.152: 20.2,5 21.2,4
S$472
  Bottom 0.152: 21.6,5 21.8,5
S$473
  Bottom 0.152: 21.8,5 22.8,4
S$474
  Bottom 0.152: 23.6,5 24.4,4.2
S$475
  Bottom 0.152: 24.4,4.2 24.4,4
S$476
  Bottom 0.152: 17.2,0 16,0
S$477
  Bottom 0.152: 16,0 15,1
S$478
  Bottom 0.152: 15,1 14.6,1
S$479
  Bottom 0.152: 50.8,-1 50.2,-1
S$480
  Bottom 0.152: 50.2,-1 49.2,0
S$481
  Bottom 0.152: 48.8,-1 48.6,-1
S$482
  Bottom 0.152: 48.6,-1 47.6,0
S$483
  Bottom 0.152: 46.8,-1 46,-0.2
S$484
  Bottom 0.152: 46,-0.2 46,0
S$485
  Bottom 0.152: 44.8,-1 44.4,-0.6
S$486
  Bottom 0.152: 44.4,-0.6 44.4,0
S$487
  Bottom 0.152: 42.8,-1 42.8,0
S$488
  Bottom 0.152: 52.8,-1 51.8,-1
S$489
  Bottom 0.152: 51.8,-1 50.8,0
S$490
  Bottom 0.152: 51.8,-5 50.8,-4
S$491
  Bottom 0.152: 50.8,-4 50,-4
S$492
  Bottom 0.152: 49.8,-5 49.4,-5
S$493
  Bottom 0.152: 49.4,-5 48.4,-4
S$494
  Bottom 0.152: 47.8,-5 46.8,-4
S$495
  Bottom 0.152: 45.8,-5 45.2,-4.4
S$496
  Bottom 0.152: 45.2,-4.4 45.2,-4
S$497
  Bottom 0.152: 43.8,-5 43.6,-4.8
S$498
  Bottom 0.152: 43.6,-4.8 43.6,-4
S$499
  Bottom 0.152: 41.8,-5 42,-4.8
S$500
  Bottom 0.152: 42,-4.8 42,-4
S$501
  Bottom 0.152: 39.8,-5 40.4,-4.4
S$502
  Bottom 0.152: 40.4,-4.4 40.4,-4
S$503
  Bottom 0.152: 37.8,-5 38.8,-4
S$504
  Bottom 0.152: 35.8,-5 36.2,-5
S$505
  Bottom 0.152: 36.2,-5 37.2,-4
S$506
  Bottom 0.152: 33.8,-5 34.6,-5
S$507
  Bottom 0.152: 34.6,-5 35.6,-4
S$508
  Bottom 0.152: 40.8,-1 41.2,-0.6
S$509
  Bottom 0.152: 41.2,-0.6 41.2,0
S$510
  Bottom 0.152: 38.8,-1 39.6,-0.2
S$511
  Bottom 0.152: 39.6,-0.2 39.6,0
S$512
  Bottom 0.152: 36.8,-1 37,-1
S$513
  Bottom 0.152: 37,-1 38,0
S$514
  Bottom 0.152: 34.8,-1 35.4,-1
S$515
  Bottom 0.152: 35.4,-1 36.4,0
S$516
  Bottom 0.152: 32.8,-3 33.8,-4
S$517
  Bottom 0.152: 33.8,-4 34.8,-4
S$518
  Bottom 0.152: 34.6,1 34,1
S$519
  Bottom 0.152: 34,1 33,0
S$520
  Bottom 0.152: 33,0 32.4,0
S$521
  Bottom 0.152: 32.6,1 31.6,0
S$522
  Bottom 0.152: 31.6,0 30.8,0
S$523
  Bottom 0.152: 30.6,1 29.6,0
S$524
  Bottom 0.152: 29.6,0 29.2,0
S$525
  Bottom 0.152: 28.6,1 27.6,0
S$526
  Bottom 0.152: 26.6,1 26,0.4
S$527
  Bottom 0.152: 26,0.4 26,0
S$528
  Bottom 0.152: 35.6,5 34.6,4
S$529
  Bottom 0.152: 34.6,4 33.2,4
S$530
  Bottom 0.152: 33.6,5 33.2,5
S$531
  Bottom 0.152: 33.2,5 32.2,4
S$532
  Bottom 0.152: 32.2,4 31.6,4
S$533
  Bottom 0.152: 31.6,5 31,5
S$534
  Bottom 0.152: 31,5 30,4
S$535
  Bottom 0.152: 29.6,5 29.4,5
S$536
  Bottom 0.152: 29.4,5 28.4,4
S$537
  Bottom 0.152: 27.6,5 26.8,4.2
S$538
  Bottom 0.152: 26.8,4.2 26.8,4
S$539
  Bottom 0.152: 34,0 35.2,0
S$540
  Bottom 0.152: 35.2,0 36.2,1
S$541
  Bottom 0.152: 36.2,1 36.6,1
S$542
  Bottom 0.8: 7.4,12.9 7.4,11.1
S$543
  Bottom 0.8: 6.4,15.1 6.4,16.9
S$544
  Bottom 0.8: 4.4,15.1 4.4,16.9
S$545
  Bottom 0.8: 3.4,12.9 3.4,11.1
S$546
  Bottom 0.8: 1.4,12.9 1.4,11.1
S$547
  Bottom 0.8: 2.4,15.1 2.4,16.9
S$548
  Bottom 0.8: 0.4,15.1 0.4,16.9
S$549
  Bottom 0.8: -0.6,12.9 -0.6,11.1
S$550
  Bottom 0.8: -2.6,12.9 -2.6,11.1
S$551
  Bottom 0.8: -1.6,15.1 -1.6,16.9
S$552
  Bottom 0.8: 17.4,12.9 17.4,11.1
S$553
  Bottom 0.8: 19.4,12.9 19.4,11.1
S$554
  Bottom 0.8: 16.4,15.1 16.4,16.9
S$555
  Bottom 0.8: 18.4,15.1 18.4,16.9
S$556
  Bottom 0.8: 13.4,12.9 13.4,11.1
S$557
  Bottom 0.8: 15.4,12.9 15.4,11.1
S$558
  Bottom 0.8: 12.4,15.1 12.4,16.9
S$559
  Bottom 0.8: 14.4,15.1 14.4,16.9
S$560
  Bottom 0.8: -7.4,20.9 -7.4,19.1
S$561
  Bottom 0.8: -5.4,20.9 -5.4,19.1
S$562
  Bottom 0.8: -8.4,23.1 -8.4,24.9
S$563
  Bottom 0.8: -6.4,23.1 -6.4,24.9
S$564
  Bottom 0.8: -11.4,20.9 -11.4,19.1
S$565
  Bottom 0.8: -9.4,20.9 -9.4,19.1
S$566
  Bottom 0.8: -10.4,23.1 -10.4,24.9
S$567
  Bottom 0.8: -12.4,23.1 -12.4,24.9
S$568
  Bottom 0.8: -13.4,20.9 -13.4,19.1
S$569
  Bottom 0.8: -15.4,20.9 -15.4,19.1
S$570
  Bottom 0.8: -14.4,23.1 -14.4,24.9
S$571
  Bottom 0.8: -16.4,23.1 -16.4,24.9
S$572
  Bottom 0.8: -17.4,20.9 -17.4,19.1
S$573
  Bottom 0.8: -19.4,20.9 -19.4,19.1
S$574
  Bottom 0.8: -18.4,23.1 -18.4,24.9
S$575
  Bottom 0.8: 0.6,20.9 0.6,19.1
S$576
  Bottom 0.8: 2.6,20.9 2.6,19.1
S$577
  Bottom 0.8: -0.4,23.1 -0.4,24.9
S$578
  Bottom 0.8: 1.6,23.1 1.6,24.9
S$579
  Bottom 0.8: -3.4,20.9 -3.4,19.1
S$580
  Bottom 0.8: -1.4,20.9 -1.4,19.1
S$581
  Bottom 0.8: -4.4,23.1 -4.4,24.9
S$582
  Bottom 0.8: -2.4,23.1 -2.4,24.9
S$583
  Bottom 0.8: -24.6,12.9 -24.6,11.1
S$584
  Bottom 0.8: -22.6,12.9 -22.6,11.1
S$585
  Bottom 0.8: -25.6,15.1 -25.6,16.9
S$586
  Bottom 0.8: -23.6,15.1 -23.6,16.9
S$587
  Bottom 0.8: -28.6,12.9 -28.6,11.1
S$588
  Bottom 0.8: -26.6,12.9 -26.6,11.1
S$589
  Bottom 0.8: -27.6,15.1 -27.6,16.9
S$590
  Bottom 0.8: -29.6,15.1 -29.6,16.9
S$591
  Bottom 0.8: -30.6,12.9 -30.6,11.1
S$592
  Bottom 0.8: -32.6,12.9 -32.6,11.1
S$593
  Bottom 0.8: -31.6,15.1 -31.6,16.9
S$594
  Bottom 0.8: -33.6,15.1 -33.6,16.9
S$595
  Bottom 0.8: -34.6,12.9 -34.6,11.1
S$596
  Bottom 0.8: -36.6,12.9 -36.6,11.1
S$597
  Bottom 0.8: -35.6,15.1 -35.6,16.9
S$598
  Bottom 0.8: -16.6,12.9 -16.6,11.1
S$599
  Bottom 0.8: -14.6,12.9 -14.6,11.1
S$600
  Bottom 0.8: -17.6,15.1 -17.6,16.9
S$601
  Bottom 0.8: -15.6,15.1 -15.6,16.9
S$602
  Bottom 0.8: -20.6,12.9 -20.6,11.1
S$603
  Bottom 0.8: -18.6,12.9 -18.6,11.1
S$604
  Bottom 0.8: -21.6,15.1 -21.6,16.9
S$605
  Bottom 0.8: -19.6,15.1 -19.6,16.9
S$606
  Bottom 0.8: 26.6,20.9 26.6,19.1
S$607
  Bottom 0.8: 28.6,20.9 28.6,19.1
S$608
  Bottom 0.8: 25.6,23.1 25.6,24.9
S$609
  Bottom 0.8: 27.6,23.1 27.6,24.9
S$610
  Bottom 0.8: 22.6,20.9 22.6,19.1
S$611
  Bottom 0.8: 24.6,20.9 24.6,19.1
S$612
  Bottom 0.8: 23.6,23.1 23.6,24.9
S$613
  Bottom 0.8: 21.6,23.1 21.6,24.9
S$614
  Bottom 0.8: 20.6,20.9 20.6,19.1
S$615
  Bottom 0.8: 18.6,20.9 18.6,19.1
S$616
  Bottom 0.8: 19.6,23.1 19.6,24.9
S$617
  Bottom 0.8: 17.6,23.1 17.6,24.9
S$618
  Bottom 0.8: 16.6,20.9 16.6,19.1
S$619
  Bottom 0.8: 14.6,20.9 14.6,19.1
S$620
  Bottom 0.8: 15.6,23.1 15.6,24.9
S$621
  Bottom 0.8: 34.6,20.9 34.6,19.1
S$622
  Bottom 0.8: 36.6,20.9 36.6,19.1
S$623
  Bottom 0.8: 33.6,23.1 33.6,24.9
S$624
  Bottom 0.8: 35.6,23.1 35.6,24.9
S$625
  Bottom 0.8: 30.6,20.9 30.6,19.1
S$626
  Bottom 0.8: 32.6,20.9 32.6,19.1
S$627
  Bottom 0.8: 29.6,23.1 29.6,24.9
S$628
  Bottom 0.8: 31.6,23.1 31.6,24.9
S$629
  Bottom 0.8: -41.8,20.9 -41.8,19.1
S$630
  Bottom 0.8: -39.8,20.9 -39.8,19.1
S$631
  Bottom 0.8: -42.8,23.1 -42.8,24.9
S$632
  Bottom 0.8: -40.8,23.1 -40.8,24.9
S$633
  Bottom 0.8: -45.8,20.9 -45.8,19.1
S$634
  Bottom 0.8: -43.8,20.9 -43.8,19.1
S$635
  Bottom 0.8: -44.8,23.1 -44.8,24.9
S$636
  Bottom 0.8: -46.8,23.1 -46.8,24.9
S$637
  Bottom 0.8: -47.8,20.9 -47.8,19.1
S$638
  Bottom 0.8: -49.8,20.9 -49.8,19.1
S$639
  Bottom 0.8: -48.8,23.1 -48.8,24.9
S$640
  Bottom 0.8: -50.8,23.1 -50.8,24.9
S$641
  Bottom 0.8: -51.8,20.9 -51.8,19.1
S$642
  Bottom 0.8: -53.8,20.9 -53.8,19.1
S$643
  Bottom 0.8: -52.8,23.1 -52.8,24.9
S$644
  Bottom 0.8: -33.8,20.9 -33.8,19.1
S$645
  Bottom 0.8: -31.8,20.9 -31.8,19.1
S$646
  Bottom 0.8: -34.8,23.1 -34.8,24.9
S$647
  Bottom 0.8: -32.8,23.1 -32.8,24.9
S$648
  Bottom 0.8: -37.8,20.9 -37.8,19.1
S$649
  Bottom 0.8: -35.8,20.9 -35.8,19.1
S$650
  Bottom 0.8: -38.8,23.1 -38.8,24.9
S$651
  Bottom 0.8: -36.8,23.1 -36.8,24.9
S$652
  Bottom 0.8: 43.8,12.9 43.8,11.1
S$653
  Bottom 0.8: 45.8,12.9 45.8,11.1
S$654
  Bottom 0.8: 42.8,15.1 42.8,16.9
S$655
  Bottom 0.8: 44.8,15.1 44.8,16.9
S$656
  Bottom 0.8: 39.8,12.9 39.8,11.1
S$657
  Bottom 0.8: 41.8,12.9 41.8,11.1
S$658
  Bottom 0.8: 40.8,15.1 40.8,16.9
S$659
  Bottom 0.8: 38.8,15.1 38.8,16.9
S$660
  Bottom 0.8: 37.8,12.9 37.8,11.1
S$661
  Bottom 0.8: 35.8,12.9 35.8,11.1
S$662
  Bottom 0.8: 36.8,15.1 36.8,16.9
S$663
  Bottom 0.8: 34.8,15.1 34.8,16.9
S$664
  Bottom 0.8: 33.8,12.9 33.8,11.1
S$665
  Bottom 0.8: 31.8,12.9 31.8,11.1
S$666
  Bottom 0.8: 32.8,15.1 32.8,16.9
S$667
  Bottom 0.8: 51.8,12.9 51.8,11.1
S$668
  Bottom 0.8: 53.8,12.9 53.8,11.1
S$669
  Bottom 0.8: 50.8,15.1 50.8,16.9
S$670
  Bottom 0.8: 52.8,15.1 52.8,16.9
S$671
  Bottom 0.8: 47.8,12.9 47.8,11.1
S$672
  Bottom 0.8: 49.8,12.9 49.8,11.1
S$673
  Bottom 0.8: 46.8,15.1 46.8,16.9
S$674
  Bottom 0.8: 48.8,15.1 48.8,16.9
S$803
  Bottom 0.152: -52.8,23 -51.8,22
S$804
  Bottom 0.152: -51.8,22 -50.8,22
S$805
  Bottom 0.152: -50.8,23 -50.2,23
S$806
  Bottom 0.152: -50.2,23 -49.2,22
S$807
  Bottom 0.152: -48.8,23 -48.6,23
S$808
  Bottom 0.152: -48.6,23 -47.6,22
S$809
  Bottom 0.152: -46.8,23 -46,22.2
S$810
  Bottom 0.152: -46,22.2 -46,22
S$811
  Bottom 0.152: -44.8,23 -44.4,22.6
S$812
  Bottom 0.152: -44.4,22.6 -44.4,22
S$813
  Bottom 0.152: -42.8,23 -42.8,22
S$814
  Bottom 0.152: -40.8,23 -41.2,22.6
S$815
  Bottom 0.152: -41.2,22.6 -41.2,22
S$816
  Bottom 0.152: -38.8,23 -39.6,22.2
S$817
  Bottom 0.152: -39.6,22.2 -39.6,22
S$818
  Bottom 0.152: -36.8,23 -37,23
S$819
  Bottom 0.152: -37,23 -38,22
S$820
  Bottom 0.152: -34.8,23 -35.4,23
S$821
  Bottom 0.152: -35.4,23 -36.4,22
S$822
  Bottom 0.152: -32.8,23 -33.8,22
S$823
  Bottom 0.152: -33.8,22 -34.8,22
S$824
  Bottom 0.152: -51.8,19 -50.8,18
S$825
  Bottom 0.152: -50.8,18 -50,18
S$826
  Bottom 0.152: -49.8,19 -48.8,18
S$827
  Bottom 0.152: -48.8,18 -48.4,18
S$828
  Bottom 0.152: -47.8,19 -46.8,18
S$829
  Bottom 0.152: -45.8,19 -45.2,18.4
S$830
  Bottom 0.152: -45.2,18.4 -45.2,18
S$831
  Bottom 0.152: -43.8,19 -43.6,18.8
S$832
  Bottom 0.152: -43.6,18.8 -43.6,18
S$833
  Bottom 0.152: -41.8,19 -42,18.8
S$834
  Bottom 0.152: -42,18.8 -42,18
S$835
  Bottom 0.152: -39.8,19 -40.4,18.4
S$836
  Bottom 0.152: -40.4,18.4 -40.4,18
S$837
  Bottom 0.152: -37.8,19 -38.8,18
S$838
  Bottom 0.152: -35.8,19 -36.8,18
S$839
  Bottom 0.152: -36.8,18 -37.2,18
S$840
  Bottom 0.152: -33.8,19 -34.8,18
S$841
  Bottom 0.152: -34.8,18 -35.6,18
S$842
  Bottom 0.152: -36.6,13 -35.6,14
S$843
  Bottom 0.152: -35.6,14 -34,14
S$844
  Bottom 0.152: -34.6,13 -33.8,13
S$845
  Bottom 0.152: -33.8,13 -32.8,14
S$846
  Bottom 0.152: -32.8,14 -32.4,14
S$847
  Bottom 0.152: -32.6,13 -31.8,13
S$848
  Bottom 0.152: -31.8,13 -30.8,14
S$849
  Bottom 0.152: -30.6,13 -30.2,13
S$850
  Bottom 0.152: -30.2,13 -29.2,14
S$851
  Bottom 0.152: -28.6,13 -27.6,14
S$852
  Bottom 0.152: -26.6,13 -26,13.6
S$853
  Bottom 0.152: -26,13.6 -26,14
S$854
  Bottom 0.152: -35.6,17 -35,17
S$855
  Bottom 0.152: -35,17 -34,18
S$856
  Bottom 0.152: -34,18 -33.2,18
S$857
  Bottom 0.152: -33.6,17 -33,17
S$858
  Bottom 0.152: -33,17 -32,18
S$859
  Bottom 0.152: -32,18 -31.6,18
S$860
  Bottom 0.152: -31.6,17 -31,17
S$861
  Bottom 0.152: -31,17 -30,18
S$862
  Bottom 0.152: -29.6,17 -29.4,17
S$863
  Bottom 0.152: -29.4,17 -28.4,18
S$864
  Bottom 0.152: -27.6,17 -26.8,17.8
S$865
  Bottom 0.152: -26.8,17.8 -26.8,18
S$866
  Bottom 0.152: 1.6,23 0.6,22
S$867
  Bottom 0.152: 0.6,22 -0.4,22
S$868
  Bottom 0.152: -0.4,23 -1,23
S$869
  Bottom 0.152: -1,23 -2,22
S$870
  Bottom 0.152: -2.4,23 -2.6,23
S$871
  Bottom 0.152: -2.6,23 -3.6,22
S$872
  Bottom 0.152: -4.4,23 -5.2,22.2
S$873
  Bottom 0.152: -5.2,22.2 -5.2,22
S$874
  Bottom 0.152: -6.4,23 -6.8,22.6
S$875
  Bottom 0.152: -6.8,22.6 -6.8,22
S$876
  Bottom 0.152: -8.4,23 -8.4,22
S$877
  Bottom 0.152: -10.4,23 -10,22.6
S$878
  Bottom 0.152: -10,22.6 -10,22
S$879
  Bottom 0.152: -12.4,23 -11.6,22.2
S$880
  Bottom 0.152: -11.6,22.2 -11.6,22
S$881
  Bottom 0.152: -14.4,23 -14.2,23
S$882
  Bottom 0.152: -14.2,23 -13.2,22
S$883
  Bottom 0.152: -16.4,23 -15.8,23
S$884
  Bottom 0.152: -15.8,23 -14.8,22
S$885
  Bottom 0.152: -18.4,23 -17.4,22
S$886
  Bottom 0.152: -17.4,22 -16.4,22
S$887
  Bottom 0.152: 0.6,19 -0.4,18
S$888
  Bottom 0.152: -0.4,18 -1.2,18
S$889
  Bottom 0.152: -1.4,19 -2.4,18
S$890
  Bottom 0.152: -2.4,18 -2.8,18
S$891
  Bottom 0.152: -3.4,19 -4.4,18
S$892
  Bottom 0.152: -5.4,19 -6,18.4
S$893
  Bottom 0.152: -6,18.4 -6,18
S$894
  Bottom 0.152: -7.4,19 -7.6,18.8
S$895
  Bottom 0.152: -7.6,18.8 -7.6,18
S$896
  Bottom 0.152: -9.4,19 -9.2,18.8
S$897
  Bottom 0.152: -9.2,18.8 -9.2,18
S$898
  Bottom 0.152: -11.4,19 -10.8,18.4
S$899
  Bottom 0.152: -10.8,18.4 -10.8,18
S$900
  Bottom 0.152: -13.4,19 -12.4,18
S$901
  Bottom 0.152: -15.4,19 -14.4,18
S$902
  Bottom 0.152: -14.4,18 -14,18
S$903
  Bottom 0.152: -17.4,19 -16.4,18
S$904
  Bottom 0.152: -16.4,18 -15.6,18
S$905
  Bottom 0.152: -14.6,13 -15.6,14
S$906
  Bottom 0.152: -15.6,14 -17.2,14
S$907
  Bottom 0.152: -16.6,13 -17.4,13
S$908
  Bottom 0.152: -17.4,13 -18.4,14
S$909
  Bottom 0.152: -18.4,14 -18.8,14
S$910
  Bottom 0.152: -18.6,13 -19.4,13
S$911
  Bottom 0.152: -19.4,13 -20.4,14
S$912
  Bottom 0.152: -20.6,13 -21,13
S$913
  Bottom 0.152: -21,13 -22,14
S$914
  Bottom 0.152: -22.6,13 -23.6,14
S$915
  Bottom 0.152: -24.6,13 -25.2,13.6
S$916
  Bottom 0.152: -25.2,13.6 -25.2,14
S$917
  Bottom 0.152: -15.6,17 -16.2,17
S$918
  Bottom 0.152: -16.2,17 -17.2,18
S$919
  Bottom 0.152: -17.2,18 -18,18
S$920
  Bottom 0.152: -17.6,17 -18.2,17
S$921
  Bottom 0.152: -18.2,17 -19.2,18
S$922
  Bottom 0.152: -19.2,18 -19.6,18
S$923
  Bottom 0.152: -19.6,17 -20.2,17
S$924
  Bottom 0.152: -20.2,17 -21.2,18
S$925
  Bottom 0.152: -21.6,17 -21.8,17
S$926
  Bottom 0.152: -21.8,17 -22.8,18
S$927
  Bottom 0.152: -23.6,17 -24.4,17.8
S$928
  Bottom 0.152: -24.4,17.8 -24.4,18
S$929
  Bottom 0.152: 0.4,17 1,17
S$930
  Bottom 0.152: 1,17 2,18
S$931
  Bottom 0.152: 2.4,17 2.6,17
S$932
  Bottom 0.152: 2.6,17 3.6,18
S$933
  Bottom 0.152: 4.4,17 5.2,17.8
S$934
  Bottom 0.152: 5.2,17.8 5.2,18
S$935
  Bottom 0.152: 6.4,17 6.8,17.4
S$936
  Bottom 0.152: 6.8,17.4 6.8,18
S$937
  Bottom 0.152: 8.4,17 8.4,18
S$938
  Bottom 0.152: -1.6,17 -0.6,17
S$939
  Bottom 0.152: -0.6,17 0.4,18
S$940
  Bottom 0.152: -0.6,13 0.4,14
S$941
  Bottom 0.152: 0.4,14 1.2,14
S$942
  Bottom 0.152: 1.4,13 1.8,13
S$943
  Bottom 0.152: 1.8,13 2.8,14
S$944
  Bottom 0.152: 3.4,13 4.4,14
S$945
  Bottom 0.152: 5.4,13 6,13.6
S$946
  Bottom 0.152: 6,13.6 6,14
S$947
  Bottom 0.152: 7.4,13 7.6,13.2
S$948
  Bottom 0.152: 7.6,13.2 7.6,14
S$949
  Bottom 0.152: 9.4,13 9.2,13.2
S$950
  Bottom 0.152: 9.2,13.2 9.2,14
S$951
  Bottom 0.152: 11.4,13 10.8,13.6
S$952
  Bottom 0.152: 10.8,13.6 10.8,14
S$953
  Bottom 0.152: 13.4,13 12.4,14
S$954
  Bottom 0.152: 15.4,13 15,13
S$955
  Bottom 0.152: 15,13 14,14
S$956
  Bottom 0.152: 17.4,13 16.6,13
S$957
  Bottom 0.152: 16.6,13 15.6,14
S$958
  Bottom 0.152: 10.4,17 10,17.4
S$959
  Bottom 0.152: 10,17.4 10,18
S$960
  Bottom 0.152: 12.4,17 11.6,17.8
S$961
  Bottom 0.152: 11.6,17.8 11.6,18
S$962
  Bottom 0.152: 14.4,17 14.2,17
S$963
  Bottom 0.152: 14.2,17 13.2,18
S$964
  Bottom 0.152: 16.4,17 15.8,17
S$965
  Bottom 0.152: 15.8,17 14.8,18
S$966
  Bottom 0.152: 18.4,15 17.4,14
S$967
  Bottom 0.152: 17.4,14 16.4,14
S$968
  Bottom 0.152: 16.6,19 17.2,19
S$969
  Bottom 0.152: 17.2,19 18.2,18
S$970
  Bottom 0.152: 18.2,18 18.8,18
S$971
  Bottom 0.152: 18.6,19 19.6,18
S$972
  Bottom 0.152: 19.6,18 20.4,18
S$973
  Bottom 0.152: 20.6,19 21.6,18
S$974
  Bottom 0.152: 21.6,18 22,18
S$975
  Bottom 0.152: 22.6,19 23.6,18
S$976
  Bottom 0.152: 24.6,19 25.2,18.4
S$977
  Bottom 0.152: 25.2,18.4 25.2,18
S$978
  Bottom 0.152: 15.6,23 16.6,22
S$979
  Bottom 0.152: 16.6,22 18,22
S$980
  Bottom 0.152: 17.6,23 18,23
S$981
  Bottom 0.152: 18,23 19,22
S$982
  Bottom 0.152: 19,22 19.6,22
S$983
  Bottom 0.152: 19.6,23 20.2,23
S$984
  Bottom 0.152: 20.2,23 21.2,22
S$985
  Bottom 0.152: 21.6,23 21.8,23
S$986
  Bottom 0.152: 21.8,23 22.8,22
S$987
  Bottom 0.152: 23.6,23 24.4,22.2
S$988
  Bottom 0.152: 24.4,22.2 24.4,22
S$989
  Bottom 0.152: 17.2,18 16,18
S$990
  Bottom 0.152: 16,18 15,19
S$991
  Top 1.778: -104.08,-3.17 -104.08,-1.65
S$992
  Top 1.778: -99,-3.17 -99,-1.65
S$993
  Top 1.778: -93.92,-3.17 -93.92,-1.65
S$994
  Bottom 0.152: 15,19 14.6,19
S$995
  Bottom 0.152: 50.8,17 50.2,17
S$996
  Bottom 0.152: 50.2,17 49.2,18
S$997
  Bottom 0.152: 48.8,17 48.6,17
S$998
  Bottom 0.152: 48.6,17 47.6,18
S$999
  Bottom 0.152: 46.8,17 46,17.8
S$1000
  Bottom 0.152: 46,17.8 46,18
S$1001
  Bottom 0.152: 44.8,17 44.4,17.4
S$1002
  Bottom 0.152: 44.4,17.4 44.4,18
S$1003
  Bottom 0.152: 42.8,17 42.8,18
S$1004
  Bottom 0.152: 52.8,17 51.8,17
S$1005
  Bottom 0.152: 51.8,17 50.8,18
S$1006
  Bottom 0.152: 51.8,13 50.8,14
S$1007
  Bottom 0.152: 50.8,14 50,14
S$1008
  Bottom 0.152: 49.8,13 49.4,13
S$1009
  Bottom 0.152: 49.4,13 48.4,14
S$1010
  Bottom 0.152: 47.8,13 46.8,14
S$1011
  Bottom 0.152: 45.8,13 45.2,13.6
S$1012
  Bottom 0.152: 45.2,13.6 45.2,14
S$1013
  Bottom 0.152: 43.8,13 43.6,13.2
S$1014
  Bottom 0.152: 43.6,13.2 43.6,14
S$1015
  Bottom 0.152: 41.8,13 42,13.2
S$1016
  Bottom 0.152: 42,13.2 42,14
S$1017
  Bottom 0.152: 39.8,13 40.4,13.6
S$1018
  Bottom 0.152: 40.4,13.6 40.4,14
S$1019
  Bottom 0.152: 37.8,13 38.8,14
S$1020
  Bottom 0.152: 35.8,13 36.2,13
S$1021
  Bottom 0.152: 36.2,13 37.2,14
S$1022
  Bottom 0.152: 33.8,13 34.6,13
S$1023
  Bottom 0.152: 34.6,13 35.6,14
S$1024
  Bottom 0.152: 40.8,17 41.2,17.4
S$1025
  Bottom 0.152: 41.2,17.4 41.2,18
S$1026
  Bottom 0.152: 38.8,17 39.6,17.8
S$1027
  Bottom 0.152: 39.6,17.8 39.6,18
S$1028
  Bottom 0.152: 36.8,17 37,17
S$1029
  Bottom 0.152: 37,17 38,18
S$1030
  Bottom 0.152: 34.8,17 35.4,17
S$1031
  Bottom 0.152: 35.4,17 36.4,18
S$1032
  Bottom 0.152: 32.8,15 33.8,14
S$1033
  Bottom 0.152: 33.8,14 34.8,14
S$1034
  Bottom 0.152: 34.6,19 34,19
S$1035
  Bottom 0.152: 34,19 33,18
S$1036
  Bottom 0.152: 33,18 32.4,18
S$1037
  Bottom 0.152: 32.6,19 31.6,18
S$1038
  Bottom 0.152: 31.6,18 30.8,18
S$1039
  Bottom 0.152: 30.6,19 29.6,18
S$1040
  Bottom 0.152: 29.6,18 29.2,18
S$1041
  Bottom 0.152: 28.6,19 27.6,18
S$1042
  Bottom 0.152: 26.6,19 26,18.4
S$1043
  Bottom 0.152: 26,18.4 26,18
S$1044
  Bottom 0.152: 35.6,23 34.6,22
S$1045
  Bottom 0.152: 34.6,22 33.2,22
S$1046
  Bottom 0.152: 33.6,23 33.2,23
S$1047
  Bottom 0.152: 33.2,23 32.2,22
S$1048
  Bottom 0.152: 32.2,22 31.6,22
S$1049
  Bottom 0.152: 31.6,23 31,23
S$1050
  Bottom 0.152: 31,23 30,22
S$1051
  Bottom 0.152: 29.6,23 29.4,23
S$1052
  Bottom 0.152: 29.4,23 28.4,22
S$1053
  Bottom 0.152: 27.6,23 26.8,22.2
S$1054
  Bottom 0.152: 26.8,22.2 26.8,22
S$1055
  Bottom 0.152: 34,18 35.2,18
S$1056
  Bottom 0.152: 35.2,18 36.2,19
S$1057
  Bottom 0.152: 36.2,19 36.6,19
S$1058  (2 unrouted)
  Top 0.813: 65,22.5 65,13.5
  Top 1.8: 66,19.5 64,19.5 | 66,22.5 65,22.5 64,22.5 | 66,16.5 64,16.5 | 66,13.5 65,13.5 64,13.5
S$1059
  Top 1.778: -104.08,14.82 -104.08,16.35
S$1060
  Top 1.778: -104.08,19.65 -104.08,21.18
S$1061
  Top 1.778: -99,14.82 -99,16.35
S$1062
  Top 1.778: -99,19.65 -99,21.18
S$1063
  Top 1.778: -93.92,14.82 -93.92,16.35
S$1064
  Top 1.778: -93.92,19.65 -93.92,21.18
S$1065
  Top 1.778: 93.92,14.82 93.92,16.35
S$1066
  Top 1.778: 93.92,19.65 93.92,21.18
S$1067
  Top 1.778: 99,14.82 99,16.35
S$1068
  Top 1.778: 99,19.65 99,21.18
S$1069
  Top 1.778: 104.08,14.82 104.08,16.35
S$1070
  Top 1.778: 104.08,19.65 104.08,21.18
S$1079
  Bottom 0.8: 9.4,30.9 9.4,29.1
S$1080
  Bottom 0.8: 11.4,30.9 11.4,29.1
S$1081
  Bottom 0.8: 8.4,33.1 8.4,34.9
S$1082
  Bottom 0.8: 10.4,33.1 10.4,34.9
S$1083
  Bottom 0.8: 5.4,30.9 5.4,29.1
S$1084
  Bottom 0.8: 7.4,30.9 7.4,29.1
S$1085
  Bottom 0.8: 6.4,33.1 6.4,34.9
S$1086
  Bottom 0.8: 4.4,33.1 4.4,34.9
S$1087
  Bottom 0.8: 3.4,30.9 3.4,29.1
S$1088
  Bottom 0.8: 1.4,30.9 1.4,29.1
S$1089
  Bottom 0.8: 2.4,33.1 2.4,34.9
S$1090
  Bottom 0.8: 0.4,33.1 0.4,34.9
S$1091
  Bottom 0.8: -0.6,30.9 -0.6,29.1
S$1092
  Bottom 0.8: -2.6,30.9 -2.6,29.1
S$1093
  Bottom 0.8: -1.6,33.1 -1.6,34.9
S$1094
  Bottom 0.8: 17.4,30.9 17.4,29.1
S$1095
  Bottom 0.8: 19.4,30.9 19.4,29.1
S$1096
  Bottom 0.8: 16.4,33.1 16.4,34.9
S$1097
  Bottom 0.8: 18.4,33.1 18.4,34.9
S$1098
  Bottom 0.8: 13.4,30.9 13.4,29.1
S$1099
  Bottom 0.8: 15.4,30.9 15.4,29.1
S$1100
  Bottom 0.8: 12.4,33.1 12.4,34.9
S$1101
  Bottom 0.8: 14.4,33.1 14.4,34.9
S$1102
  Bottom 0.8: -7.4,38.9 -7.4,37.1
S$1103
  Bottom 0.8: -5.4,38.9 -5.4,37.1
S$1104
  Bottom 0.8: -8.4,41.1 -8.4,42.9
S$1105
  Bottom 0.8: -6.4,41.1 -6.4,42.9
S$1106
  Bottom 0.8: -11.4,38.9 -11.4,37.1
S$1107
  Bottom 0.8: -9.4,38.9 -9.4,37.1
S$1108
  Bottom 0.8: -10.4,41.1 -10.4,42.9
S$1109
  Bottom 0.8: -12.4,41.1 -12.4,42.9
S$1110
  Bottom 0.8: -13.4,38.9 -13.4,37.1
S$1111
  Bottom 0.8: -15.4,38.9 -15.4,37.1
S$1112
  Bottom 0.8: -14.4,41.1 -14.4,42.9
S$1113
  Bottom 0.8: -16.4,41.1 -16.4,42.9
S$1114
  Bottom 0.8: -17.4,38.9 -17.4,37.1
S$1115
  Bottom 0.8: -19.4,38.9 -19.4,37.1
S$1116
  Bottom 0.8: -18.4,41.1 -18.4,42.9
S$1117
  Bottom 0.8: 0.6,38.9 0.6,37.1
S$1118
  Bottom 0.8: 2.6,38.9 2.6,37.1
S$1119
  Bottom 0.8: -0.4,41.1 -0.4,42.9
S$1120
  Bottom 0.8: 1.6,41.1 1.6,42.9
S$1121
  Bottom 0.8: -3.4,38.9 -3.4,37.1
S$1122
  Bottom 0.8: -1.4,38.9 -1.4,37.1
S$1123
  Bottom 0.8: -4.4,41.1 -4.4,42.9
S$1124
  Bottom 0.8: -2.4,41.1 -2.4,42.9
S$1125
  Bottom 0.8: -24.6,30.9 -24.6,29.1
S$1126
  Bottom 0.8: -22.6,30.9 -22.6,29.1
S$1127
  Bottom 0.8: -25.6,33.1 -25.6,34.9
S$1128
  Bottom 0.8: -23.6,33.1 -23.6,34.9
S$1129
  Bottom 0.8: -28.6,30.9 -28.6,29.1
S$1130
  Bottom 0.8: -26.6,30.9 -26.6,29.1
S$1131
  Bottom 0.8: -27.6,33.1 -27.6,34.9
S$1132
  Bottom 0.8: -29.6,33.1 -29.6,34.9
S$1133
  Bottom 0.8: -30.6,30.9 -30.6,29.1
S$1134
  Bottom 0.8: -32.6,30.9 -32.6,29.1
S$1135
  Bottom 0.8: -31.6,33.1 -31.6,34.9
S$1136
  Bottom 0.8: -33.6,33.1 -33.6,34.9
S$1137
  Bottom 0.8: -34.6,30.9 -34.6,29.1
S$1138
  Bottom 0.8: -36.6,30.9 -36.6,29.1
S$1139
  Bottom 0.8: -35.6,33.1 -35.6,34.9
S$1140
  Bottom 0.8: -16.6,30.9 -16.6,29.1
S$1141
  Bottom 0.8: -14.6,30.9 -14.6,29.1
S$1142
  Bottom 0.8: -17.6,33.1 -17.6,34.9
S$1143
  Bottom 0.8: -15.6,33.1 -15.6,34.9
S$1144
  Bottom 0.8: -20.6,30.9 -20.6,29.1
S$1145
  Bottom 0.8: -18.6,30.9 -18.6,29.1
S$1146
  Bottom 0.8: -21.6,33.1 -21.6,34.9
S$1147
  Bottom 0.8: -19.6,33.1 -19.6,34.9
S$1148
  Bottom 0.8: 26.6,38.9 26.6,37.1
S$1149
  Bottom 0.8: 28.6,38.9 28.6,37.1
S$1150
  Bottom 0.8: 25.6,41.1 25.6,42.9
S$1151
  Bottom 0.8: 27.6,41.1 27.6,42.9
S$1152
  Bottom 0.8: 22.6,38.9 22.6,37.1
S$1153
  Bottom 0.8: 24.6,38.9 24.6,37.1
S$1154
  Bottom 0.8: 23.6,41.1 23.6,42.9
S$1155
  Bottom 0.8: 21.6,41.1 21.6,42.9
S$1156
  Bottom 0.8: 20.6,38.9 20.6,37.1
S$1157
  Bottom 0.8: 18.6,38.9 18.6,37.1
S$1158
  Bottom 0.8: 19.6,41.1 19.6,42.9
S$1159
  Bottom 0.8: 17.6,41.1 17.6,42.9
S$1160
  Bottom 0.8: 16.6,38.9 16.6,37.1
S$1161
  Bottom 0.8: 14.6,38.9 14.6,37.1
S$1162
  Bottom 0.8: 15.6,41.1 15.6,42.9
S$1163
  Bottom 0.8: 34.6,38.9 34.6,37.1
S$1164
  Bottom 0.8: 36.6,38.9 36.6,37.1
S$1165
  Bottom 0.8: 33.6,41.1 33.6,42.9
S$1166
  Bottom 0.8: 35.6,41.1 35.6,42.9
S$1167
  Bottom 0.8: 30.6,38.9 30.6,37.1
S$1168
  Bottom 0.8: 32.6,38.9 32.6,37.1
S$1169
  Bottom 0.8: 29.6,41.1 29.6,42.9
S$1170
  Bottom 0.8: 31.6,41.1 31.6,42.9
S$1171
  Bottom 0.8: -41.8,38.9 -41.8,37.1
S$1172
  Bottom 0.8: -39.8,38.9 -39.8,37.1
S$1173
  Bottom 0.8: -42.8,41.1 -42.8,42.9
S$1174
  Bottom 0.8: -40.8,41.1 -40.8,42.9
S$1175
  Bottom 0.8: -45.8,38.9 -45.8,37.1
S$1176
  Bottom 0.8: -43.8,38.9 -43.8,37.1
S$1177
  Bottom 0.8: -44.8,41.1 -44.8,42.9
S$1178
  Bottom 0.8: -46.8,41.1 -46.8,42.9
S$1179
  Bottom 0.8: -47.8,38.9 -47.8,37.1
S$1180
  Bottom 0.8: -49.8,38.9 -49.8,37.1
S$1181
  Bottom 0.8: -48.8,41.1 -48.8,42.9
S$1182
  Bottom 0.8: -50.8,41.1 -50.8,42.9
S$1183
  Bottom 0.8: -51.8,38.9 -51.8,37.1
S$1184
  Bottom 0.8: -53.8,38.9 -53.8,37.1
S$1185
  Bottom 0.8: -52.8,41.1 -52.8,42.9
S$1186
  Bottom 0.8: -33.8,38.9 -33.8,37.1
S$1187
  Bottom 0.8: -31.8,38.9 -31.8,37.1
S$1188
  Bottom 0.8: -34.8,41.1 -34.8,42.9
S$1189
  Bottom 0.8: -32.8,41.1 -32.8,42.9
S$1190
  Bottom 0.8: -37.8,38.9 -37.8,37.1
S$1191
  Bottom 0.8: -35.8,38.9 -35.8,37.1
S$1192
  Bottom 0.8: -38.8,41.1 -38.8,42.9
S$1193
  Bottom 0.8: -36.8,41.1 -36.8,42.9
S$1194
  Bottom 0.8: 43.8,30.9 43.8,29.1
S$1195
  Bottom 0.8: 45.8,30.9 45.8,29.1
S$1196
  Bottom 0.8: 42.8,33.1 42.8,34.9
S$1197
  Bottom 0.8: 44.8,33.1 44.8,34.9
S$1198
  Bottom 0.8: 39.8,30.9 39.8,29.1
S$1199
  Bottom 0.8: 41.8,30.9 41.8,29.1
S$1200
  Bottom 0.8: 40.8,33.1 40.8,34.9
S$1201
  Bottom 0.8: 38.8,33.1 38.8,34.9
S$1202
  Bottom 0.8: 37.8,30.9 37.8,29.1
S$1203
  Bottom 0.8: 35.8,30.9 35.8,29.1
S$1204
  Bottom 0.8: 36.8,33.1 36.8,34.9
S$1205
  Bottom 0.8: 34.8,33.1 34.8,34.9
S$1206
  Bottom 0.8: 33.8,30.9 33.8,29.1
S$1207
  Bottom 0.8: 31.8,30.9 31.8,29.1
S$1208
  Bottom 0.8: 32.8,33.1 32.8,34.9
S$1209
  Bottom 0.8: 51.8,30.9 51.8,29.1
S$1210
  Bottom 0.8: 53.8,30.9 53.8,29.1
S$1211
  Bottom 0.8: 50.8,33.1 50.8,34.9
S$1212
  Bottom 0.8: 52.8,33.1 52.8,34.9
S$1213
  Bottom 0.8: 47.8,30.9 47.8,29.1
S$1214
  Bottom 0.8: 49.8,30.9 49.8,29.1
S$1215
  Bottom 0.8: 46.8,33.1 46.8,34.9
S$1216
  Bottom 0.8: 48.8,33.1 48.8,34.9
S$1345
  Bottom 0.152: -52.8,41 -51.8,40
S$1346
  Bottom 0.152: -51.8,40 -50.8,40
S$1347
  Bottom 0.152: -50.8,41 -50.2,41
S$1348
  Bottom 0.152: -50.2,41 -49.2,40
S$1349
  Bottom 0.152: -48.8,41 -48.6,41
S$1350
  Bottom 0.152: -48.6,41 -47.6,40
S$1351
  Bottom 0.152: -46.8,41 -46,40.2
S$1352
  Bottom 0.152: -46,40.2 -46,40
S$1353
  Bottom 0.152: -44.8,41 -44.4,40.6
S$1354
  Bottom 0.152: -44.4,40.6 -44.4,40
S$1355
  Bottom 0.152: -42.8,41 -42.8,40
S$1356
  Bottom 0.152: -40.8,41 -41.2,40.6
S$1357
  Bottom 0.152: -41.2,40.6 -41.2,40
S$1358
  Bottom 0.152: -38.8,41 -39.6,40.2
S$1359
  Bottom 0.152: -39.6,40.2 -39.6,40
S$1360
  Bottom 0.152: -36.8,41 -37,41
S$1361
  Bottom 0.152: -37,41 -38,40
S$1362
  Bottom 0.152: -34.8,41 -35.4,41
S$1363
  Bottom 0.152: -35.4,41 -36.4,40
S$1364
  Bottom 0.152: -32.8,41 -33.8,40
S$1365
  Bottom 0.152: -33.8,40 -34.8,40
S$1366
  Bottom 0.152: -51.8,37 -50.8,36
S$1367
  Bottom 0.152: -50.8,36 -50,36
S$1368
  Bottom 0.152: -49.8,37 -48.8,36
S$1369
  Bottom 0.152: -48.8,36 -48.4,36
S$1370
  Bottom 0.152: -47.8,37 -46.8,36
S$1371
  Bottom 0.152: -45.8,37 -45.2,36.4
S$1372
  Bottom 0.152: -45.2,36.4 -45.2,36
S$1373
  Bottom 0.152: -43.8,37 -43.6,36.8
S$1374
  Bottom 0.152: -43.6,36.8 -43.6,36
S$1375
  Bottom 0.152: -41.8,37 -42,36.8
S$1376
  Bottom 0.152: -42,36.8 -42,36
S$1377
  Bottom 0.152: -39.8,37 -40.4,36.4
S$1378
  Bottom 0.152: -40.4,36.4 -40.4,36
S$1379
  Bottom 0.152: -37.8,37 -38.8,36
S$1380
  Bottom 0.152: -35.8,37 -36.8,36
S$1381
  Bottom 0.152: -36.8,36 -37.2,36
S$1382
  Bottom 0.152: -33.8,37 -34.8,36
S$1383
  Bottom 0.152: -34.8,36 -35.6,36
S$1384
  Bottom 0.152: -36.6,31 -35.6,32
S$1385
  Bottom 0.152: -35.6,32 -34,32
S$1386
  Bottom 0.152: -34.6,31 -33.8,31
S$1387
  Bottom 0.152: -33.8,31 -32.8,32
S$1388
  Bottom 0.152: -32.8,32 -32.4,32
S$1389
  Bottom 0.152: -32.6,31 -31.8,31
S$1390
  Bottom 0.152: -31.8,31 -30.8,32
S$1391
  Bottom 0.152: -30.6,31 -30.2,31
S$1392
  Bottom 0.152: -30.2,31 -29.2,32
S$1393
  Bottom 0.152: -28.6,31 -27.6,32
S$1394
  Bottom 0.152: -26.6,31 -26,31.6
S$1395
  Bottom 0.152: -26,31.6 -26,32
S$1396
  Bottom 0.152: -35.6,35 -35,35
S$1397
  Bottom 0.152: -35,35 -34,36
S$1398
  Bottom 0.152: -34,36 -33.2,36
S$1399
  Bottom 0.152: -33.6,35 -33,35
S$1400
  Bottom 0.152: -33,35 -32,36
S$1401
  Bottom 0.152: -32,36 -31.6,36
S$1402
  Bottom 0.152: -31.6,35 -31,35
S$1403
  Bottom 0.152: -31,35 -30,36
S$1404
  Bottom 0.152: -29.6,35 -29.4,35
S$1405
  Bottom 0.152: -29.4,35 -28.4,36
S$1406
  Bottom 0.152: -27.6,35 -26.8,35.8
S$1407
  Bottom 0.152: -26.8,35.8 -26.8,36
S$1408
  Bottom 0.152: 1.6,41 0.6,40
S$1409
  Bottom 0.152: 0.6,40 -0.4,40
S$1410
  Bottom 0.152: -0.4,41 -1,41
S$1411
  Bottom 0.152: -1,41 -2,40
S$1412
  Bottom 0.152: -2.4,41 -2.6,41
S$1413
  Bottom 0.152: -2.6,41 -3.6,40
S$1414
  Bottom 0.152: -4.4,41 -5.2,40.2
S$1415
  Bottom 0.152: -5.2,40.2 -5.2,40
S$1416
  Bottom 0.152: -6.4,41 -6.8,40.6
S$1417
  Bottom 0.152: -6.8,40.6 -6.8,40
S$1418
  Bottom 0.152: -8.4,41 -8.4,40
S$1419
  Bottom 0.152: -10.4,41 -10,40.6
S$1420
  Bottom 0.152: -10,40.6 -10,40
S$1421
  Bottom 0.152: -12.4,41 -11.6,40.2
S$1422
  Bottom 0.152: -11.6,40.2 -11.6,40
S$1423
  Bottom 0.152: -14.4,41 -14.2,41
S$1424
  Bottom 0.152: -14.2,41 -13.2,40
S$1425
  Bottom 0.152: -16.4,41 -15.8,41
S$1426
  Bottom 0.152: -15.8,41 -14.8,40
S$1427
  Bottom 0.152: -18.4,41 -17.4,40
S$1428
  Bottom 0.152: -17.4,40 -16.4,40
S$1429
  Bottom 0.152: 0.6,37 -0.4,36
S$1430
  Bottom 0.152: -0.4,36 -1.2,36
S$1431
  Bottom 0.152: -1.4,37 -2.4,36
S$1432
  Bottom 0.152: -2.4,36 -2.8,36
S$1433
  Bottom 0.152: -3.4,37 -4.4,36
S$1434
  Bottom 0.152: -5.4,37 -6,36.4
S$1435
  Bottom 0.152: -6,36.4 -6,36
S$1436
  Bottom 0.152: -7.4,37 -7.6,36.8
S$1437
  Bottom 0.152: -7.6,36.8 -7.6,36
S$1438
  Bottom 0.152: -9.4,37 -9.2,36.8
S$1439
  Bottom 0.152: -9.2,36.8 -9.2,36
S$1440
  Bottom 0.152: -11.4,37 -10.8,36.4
S$1441
  Bottom 0.152: -10.8,36.4 -10.8,36
S$1442
  Bottom 0.152: -13.4,37 -12.4,36
S$1443
  Bottom 0.152: -15.4,37 -14.4,36
S$1444
  Bottom 0.152: -14.4,36 -14,36
S$1445
  Bottom 0.152: -17.4,37 -16.4,36
S$1446
  Bottom 0.152: -16.4,36 -15.6,36
S$1447
  Bottom 0.152: -14.6,31 -15.6,32
S$1448
  Bottom 0.152: -15.6,32 -17.2,32
S$1449
  Bottom 0.152: -16.6,31 -17.4,31
S$1450
  Bottom 0.152: -17.4,31 -18.4,32
S$1451
  Bottom 0.152: -18.4,32 -18.8,32
S$1452
  Bottom 0.152: -18.6,31 -19.4,31
S$1453
  Bottom 0.152: -19.4,31 -20.4,32
S$1454
  Bottom 0.152: -20.6,31 -21,31
S$1455
  Bottom 0.152: -21,31 -22,32
S$1456
  Bottom 0.152: -22.6,31 -23.6,32
S$1457
  Bottom 0.152: -24.6,31 -25.2,31.6
S$1458
  Bottom 0.152: -25.2,31.6 -25.2,32
S$1459
  Bottom 0.152: -15.6,35 -16.2,35
S$1460
  Bottom 0.152: -16.2,35 -17.2,36
S$1461
  Bottom 0.152: -17.2,36 -18,36
S$1462
  Bottom 0.152: -17.6,35 -18.2,35
S$1463
  Bottom 0.152: -18.2,35 -19.2,36
S$1464
  Bottom 0.152: -19.2,36 -19.6,36
S$1465
  Bottom 0.152: -19.6,35 -20.2,35
S$1466
  Bottom 0.152: -20.2,35 -21.2,36
S$1467
  Bottom 0.152: -21.6,35 -21.8,35
S$1468
  Bottom 0.152: -21.8,35 -22.8,36
S$1469
  Bottom 0.152: -23.6,35 -24.4,35.8
S$1470
  Bottom 0.152: -24.4,35.8 -24.4,36
S$1471
  Bottom 0.152: 0.4,35 1,35
S$1472
  Bottom 0.152: 1,35 2,36
S$1473
  Bottom 0.152: 2.4,35 2.6,35
S$1474
  Bottom 0.152: 2.6,35 3.6,36
S$1475
  Bottom 0.152: 4.4,35 5.2,35.8
S$1476
  Bottom 0.152: 5.2,35.8 5.2,36
S$1477
  Bottom 0.152: 6.4,35 6.8,35.4
S$1478
  Bottom 0.152: 6.8,35.4 6.8,36
S$1479
  Bottom 0.152: 8.4,35 8.4,36
S$1480
  Bottom 0.152: -1.6,35 -0.6,35
S$1481
  Bottom 0.152: -0.6,35 0.4,36
S$1482
  Bottom 0.152: -0.6,31 0.4,32
S$1483
  Bottom 0.152: 0.4,32 1.2,32
S$1484
  Bottom 0.152: 1.4,31 1.8,31
S$1485
  Bottom 0.152: 1.8,31 2.8,32
S$1486
  Bottom 0.152: 3.4,31 4.4,32
S$1487
  Bottom 0.152: 5.4,31 6,31.6
S$1488
  Bottom 0.152: 6,31.6 6,32
S$1489
  Bottom 0.152: 7.4,31 7.6,31.2
S$1490
  Bottom 0.152: 7.6,31.2 7.6,32
S$1491
  Bottom 0.152: 9.4,31 9.2,31.2
S$1492
  Bottom 0.152: 9.2,31.2 9.2,32
S$1493
  Bottom 0.152: 11.4,31 10.8,31.6
S$1494
  Bottom 0.152: 10.8,31.6 10.8,32
S$1495
  Bottom 0.152: 13.4,31 12.4,32
S$1496
  Bottom 0.152: 15.4,31 15,31
S$1497
  Bottom 0.152: 15,31 14,32
S$1498
  Bottom 0.152: 17.4,31 16.6,31
S$1499
  Bottom 0.152: 16.6,31 15.6,32
S$1500
  Bottom 0.152: 10.4,35 10,35.4
S$1501
  Bottom 0.152: 10,35.4 10,36
S$1502
  Bottom 0.152: 12.4,35 11.6,35.8
S$1503
  Bottom 0.152: 11.6,35.8 11.6,36
S$1504
  Bottom 0.152: 14.4,35 14.2,35
S$1505
  Bottom 0.152: 14.2,35 13.2,36
S$1506
  Bottom 0.152: 16.4,35 15.8,35
S$1507
  Bottom 0.152: 15.8,35 14.8,36
S$1508
  Bottom 0.152: 18.4,33 17.4,32
S$1509
  Bottom 0.152: 17.4,32 16.4,32
S$1510
  Bottom 0.152: 16.6,37 17.2,37
S$1511
  Bottom 0.152: 17.2,37 18.2,36
S$1512
  Bottom 0.152: 18.2,36 18.8,36
S$1513
  Bottom 0.152: 18.6,37 19.6,36
S$1514
  Bottom 0.152: 19.6,36 20.4,36
S$1515
  Bottom 0.152: 20.6,37 21.6,36
S$1516
  Bottom 0.152: 21.6,36 22,36
S$1517
  Bottom 0.152: 22.6,37 23.6,36
S$1518
  Bottom 0.152: 24.6,37 25.2,36.4
S$1519
  Bottom 0.152: 25.2,36.4 25.2,36
S$1520
  Bottom 0.152: 15.6,41 16.6,40
S$1521
  Bottom 0.152: 16.6,40 18,40
S$1522
  Bottom 0.152: 17.6,41 18,41
S$1523
  Bottom 0.152: 18,41 19,40
S$1524
  Bottom 0.152: 19,40 19.6,40
S$1525
  Bottom 0.152: 19.6,41 20.2,41
S$1526
  Bottom 0.152: 20.2,41 21.2,40
S$1527
  Bottom 0.152: 21.6,41 21.8,41
S$1528
  Bottom 0.152: 21.8,41 22.8,40
S$1529
  Bottom 0.152: 23.6,41 24.4,40.2
S$1530
  Bottom 0.152: 24.4,40.2 24.4,40
S$1531
  Bottom 0.152: 17.2,36 16,36
S$1532
  Bottom 0.152: 16,36 15,37
S$1533
  Bottom 0.152: 15,37 14.6,37
S$1534
  Bottom 0.152: 50.8,35 50.2,35
S$1535
  Bottom 0.152: 50.2,35 49.2,36
S$1536
  Bottom 0.152: 48.8,35 48.6,35
S$1537
  Bottom 0.152: 48.6,35 47.6,36
S$1538
  Bottom 0.152: 46.8,35 46,35.8
S$1539
  Bottom 0.152: 46,35.8 46,36
S$1540
  Bottom 0.152: 44.8,35 44.4,35.4
S$1541
  Bottom 0.152: 44.4,35.4 44.4,36
S$1542
  Bottom 0.152: 42.8,35 42.8,36
S$1543
  Bottom 0.152: 52.8,35 51.8,35
S$1544
  Bottom 0.152: 51.8,35 50.8,36
S$1545
  Bottom 0.152: 51.8,31 50.8,32
S$1546
  Bottom 0.152: 50.8,32 50,32
S$1547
